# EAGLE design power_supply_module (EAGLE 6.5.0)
AUTHOR: N. Jackson; REV: A; TITLE: Power Supply Module

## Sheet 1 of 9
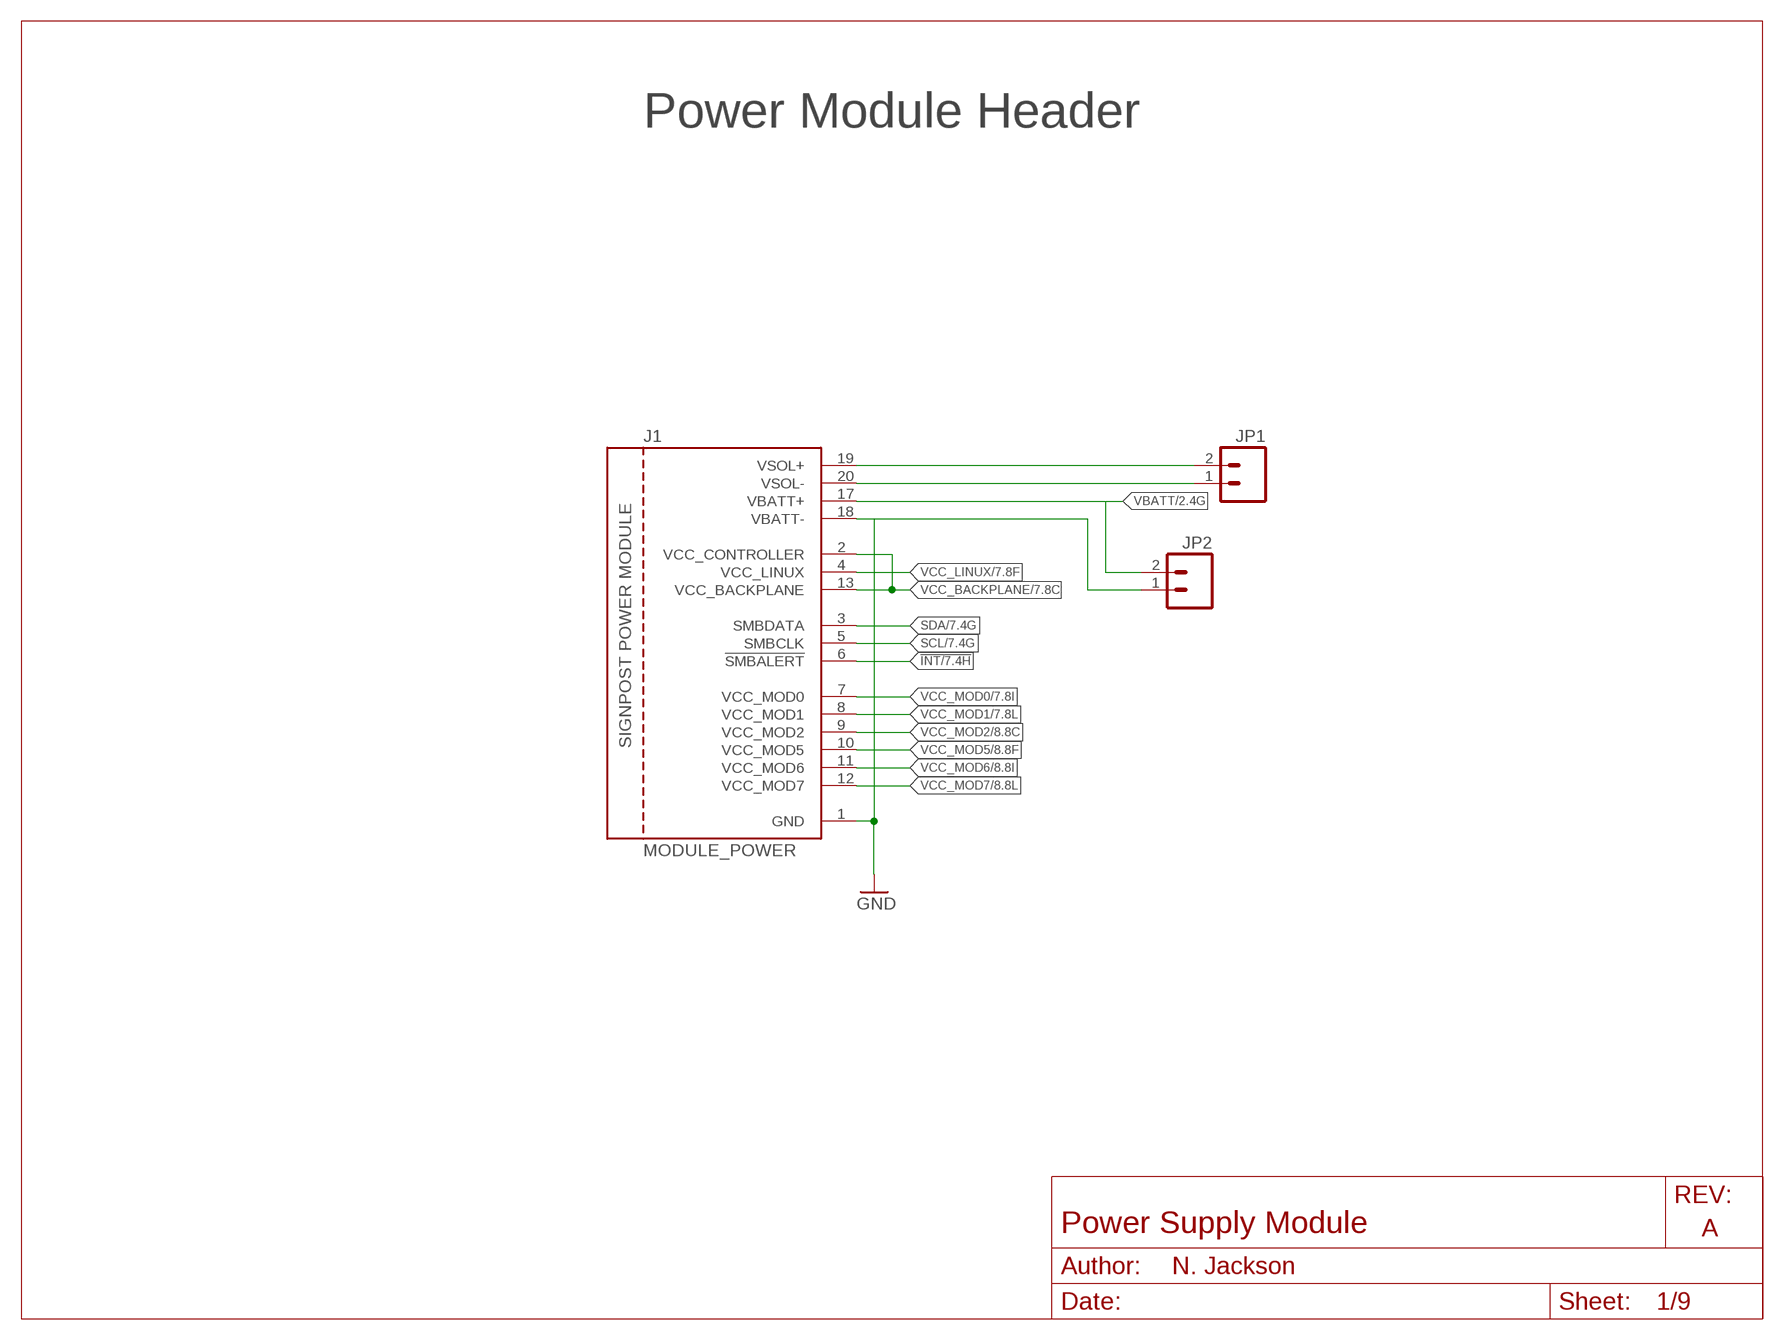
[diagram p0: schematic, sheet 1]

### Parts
J1  MODULE_POWER  [MODULE_POWER]
JP1  M02PTH  [1X02]
JP2  M02PTH  [1X02]

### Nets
!INT: J1.6(!SMBALERT) ; also sheet 7,8,9
GND: J1.1(GND) J1.18(VBATT-) JP2.1 ; also sheet 2,3,4,5,6,7,8,9
SCL: J1.5(SMBCLK) ; also sheet 7,8,9
SDA: J1.3(SMBDATA) ; also sheet 7,8,9
VBATT: J1.17(VBATT+) JP2.2 ; also sheet 2,3,4,5,6,9
VCC_BACKPLANE: J1.2(VCC_CONTROLLER) J1.13(VCC_BACKPLANE) ; also sheet 7,8,9
VCC_LINUX: J1.4(VCC_LINUX) ; also sheet 7,9
VCC_MOD0: J1.7(VCC_MOD0) ; also sheet 7,9
VCC_MOD1: J1.8(VCC_MOD1) ; also sheet 7,9
VCC_MOD2: J1.9(VCC_MOD2) ; also sheet 8,9
VCC_MOD5: J1.10(VCC_MOD5) ; also sheet 8,9
VCC_MOD6: J1.11(VCC_MOD6) ; also sheet 8,9
VCC_MOD7: J1.12(VCC_MOD7) ; also sheet 8,9
VSOL+: J1.19(VSOL+) JP1.2 ; also sheet 9
VSOL-: J1.20(VSOL-) JP1.1 ; also sheet 9

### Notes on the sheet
- Power Module Header

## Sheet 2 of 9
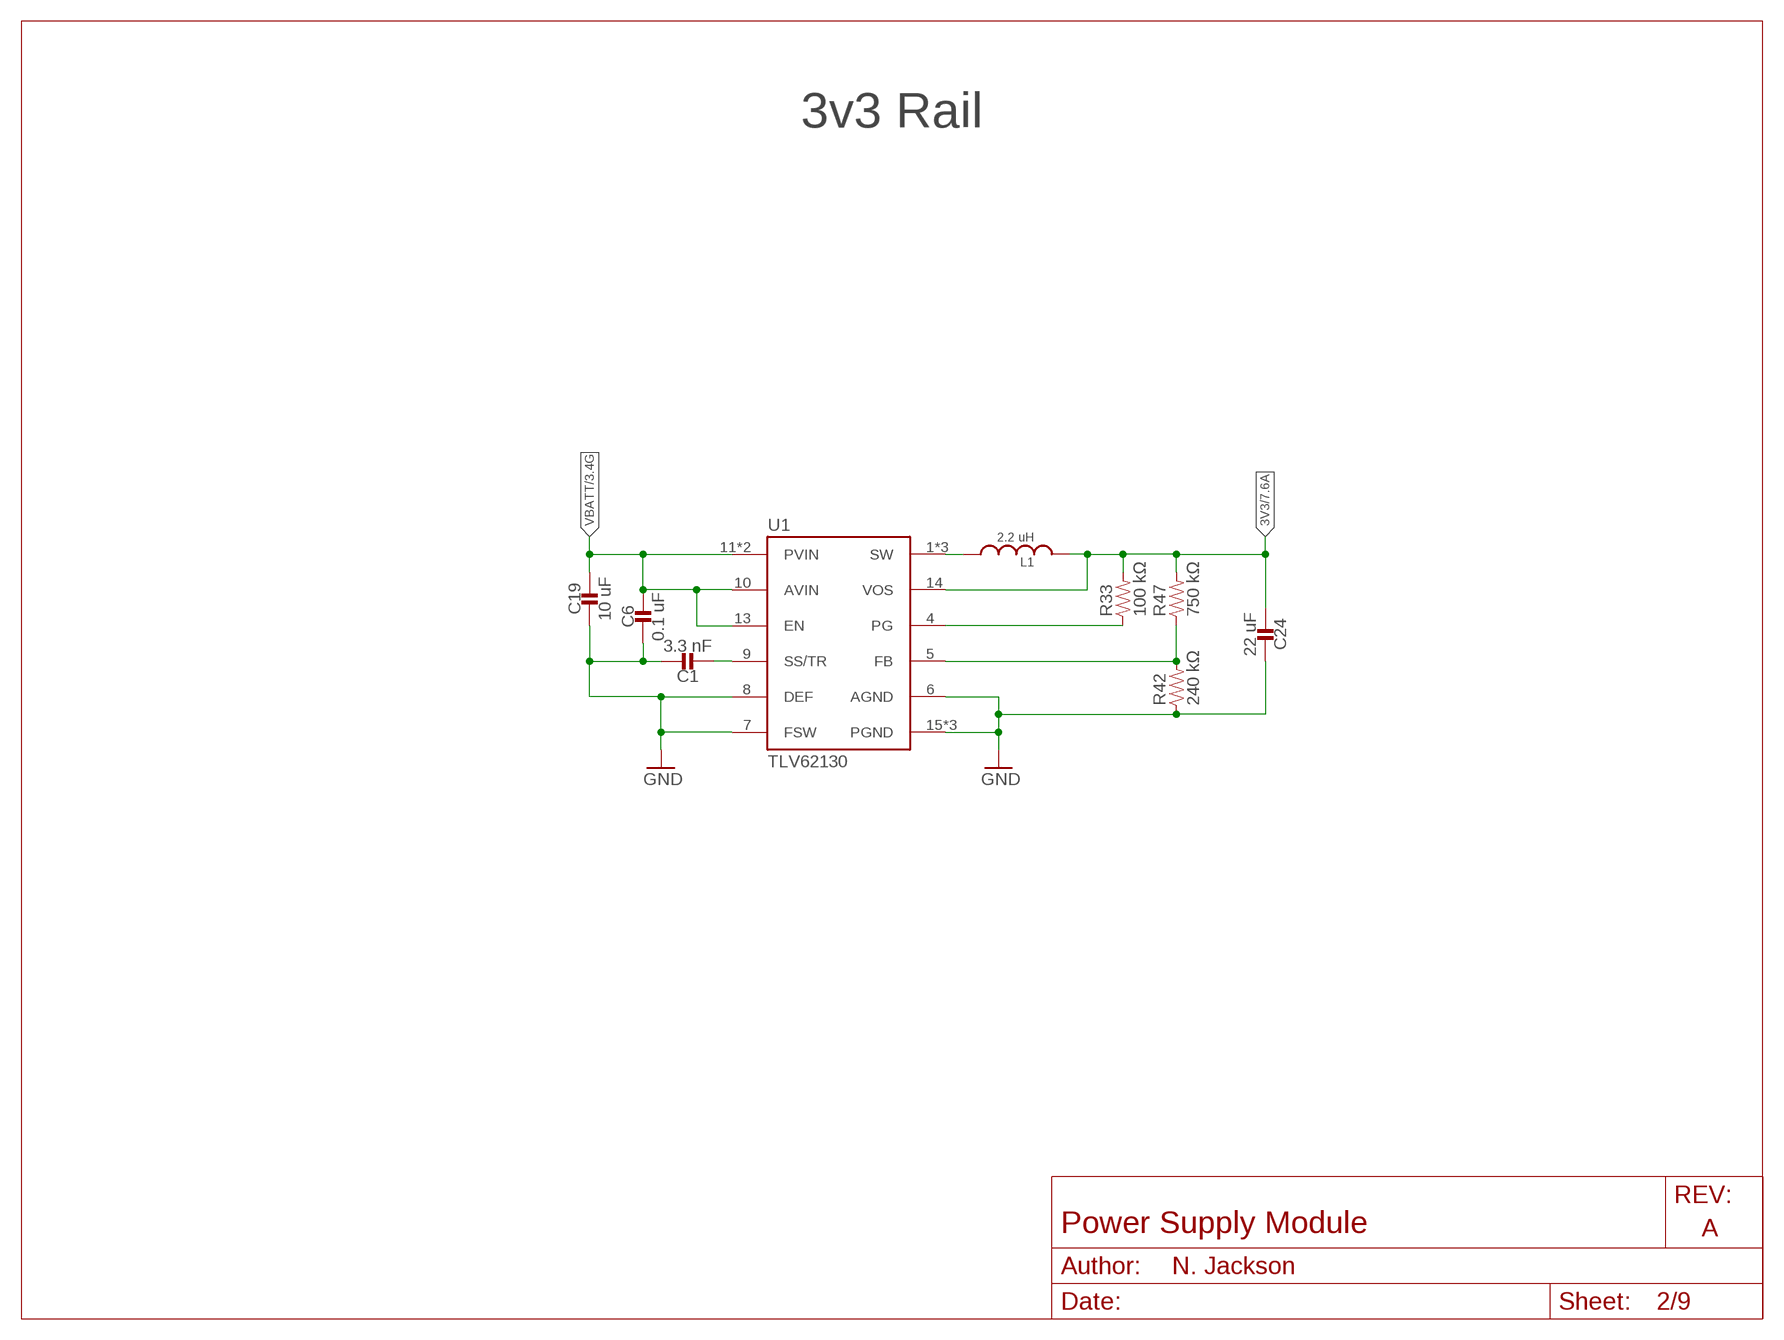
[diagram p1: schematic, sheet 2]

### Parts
C1  3.3 nF  CAPACITOR0402_CAP  [0402_CAP]
C6  0.1 uF  CAPACITOR0402_CAP  [0402_CAP]
C19  10 uF  CAPACITOR0805_CAP  [0805_CAP]
C24  22 uF  CAPACITOR0603_CAP  [0603_CAP]
L1  2.2 uH  INDUCTORIHL  [IHL-1212BZ-11]
R33  100 kΩ  RESISTOR0402_RES  [0402_RES]
R42  240 kΩ  RESISTOR0402_RES  [0402_RES]
R47  750 kΩ  RESISTOR0402_RES  [0402_RES]
U1  TLV62130  [TQFN-16/3MM]

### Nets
3V3: C24.2 L1.P$2 R33.2 R47.2 U1.14(VOS) ; also sheet 7,9
GND: C1.1 C6.2 C19.P$2 C24.1 R42.1 U1.6(AGND) U1.7(FSW) U1.8(DEF) U1.15(PGND) U1.16(PGND) U1.GND ; also sheet 1,3,4,5,6,7,8,9
N$61: C1.2 U1.9(SS/TR)
N$62: L1.P$1 U1.1(SW) U1.2(SW) U1.3(SW)
N$63: R33.1 U1.4(PG)
N$64: R42.2 R47.1 U1.5(FB)
VBATT: C6.1 C19.P$1 U1.10(AVIN) U1.11(PVIN) U1.12(PVIN) U1.13(EN) ; also sheet 1,3,4,5,6,9

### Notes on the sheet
- 3v3 Rail

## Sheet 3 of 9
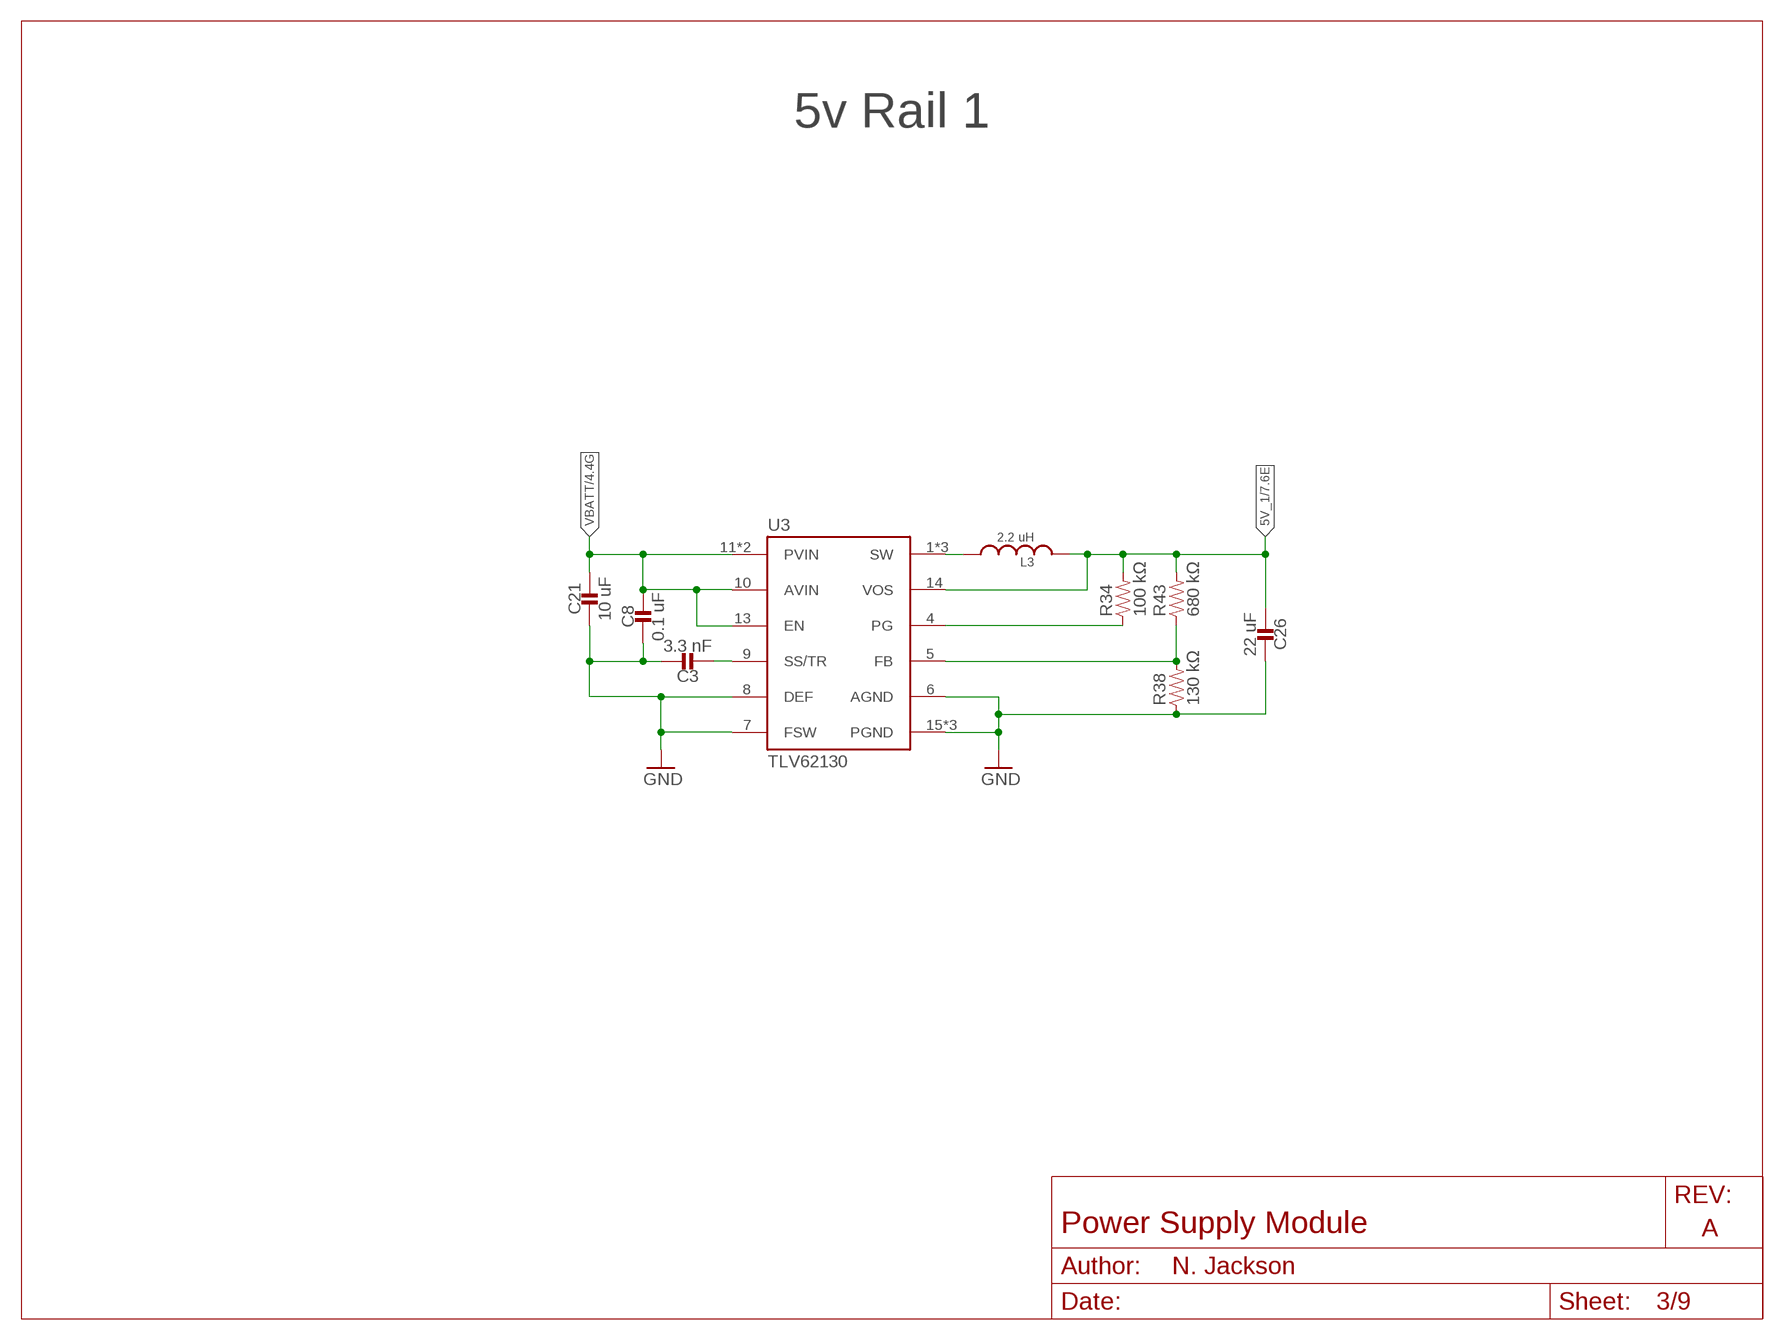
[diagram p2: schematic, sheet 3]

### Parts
C3  3.3 nF  CAPACITOR0402_CAP  [0402_CAP]
C8  0.1 uF  CAPACITOR0402_CAP  [0402_CAP]
C21  10 uF  CAPACITOR0805_CAP  [0805_CAP]
C26  22 uF  CAPACITOR0603_CAP  [0603_CAP]
L3  2.2 uH  INDUCTORIHL  [IHL-1212BZ-11]
R34  100 kΩ  RESISTOR0402_RES  [0402_RES]
R38  130 kΩ  RESISTOR0402_RES  [0402_RES]
R43  680 kΩ  RESISTOR0402_RES  [0402_RES]
U3  TLV62130  [TQFN-16/3MM]

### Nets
5V_1: C26.2 L3.P$2 R34.2 R43.2 U3.14(VOS) ; also sheet 7,9
GND: C3.1 C8.2 C21.P$2 C26.1 R38.1 U3.6(AGND) U3.7(FSW) U3.8(DEF) U3.15(PGND) U3.16(PGND) U3.GND ; also sheet 1,2,4,5,6,7,8,9
N$5: C3.2 U3.9(SS/TR)
N$6: L3.P$1 U3.1(SW) U3.2(SW) U3.3(SW)
N$7: R34.1 U3.4(PG)
N$9: R38.2 R43.1 U3.5(FB)
VBATT: C8.1 C21.P$1 U3.10(AVIN) U3.11(PVIN) U3.12(PVIN) U3.13(EN) ; also sheet 1,2,4,5,6,9

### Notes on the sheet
- 5v Rail 1

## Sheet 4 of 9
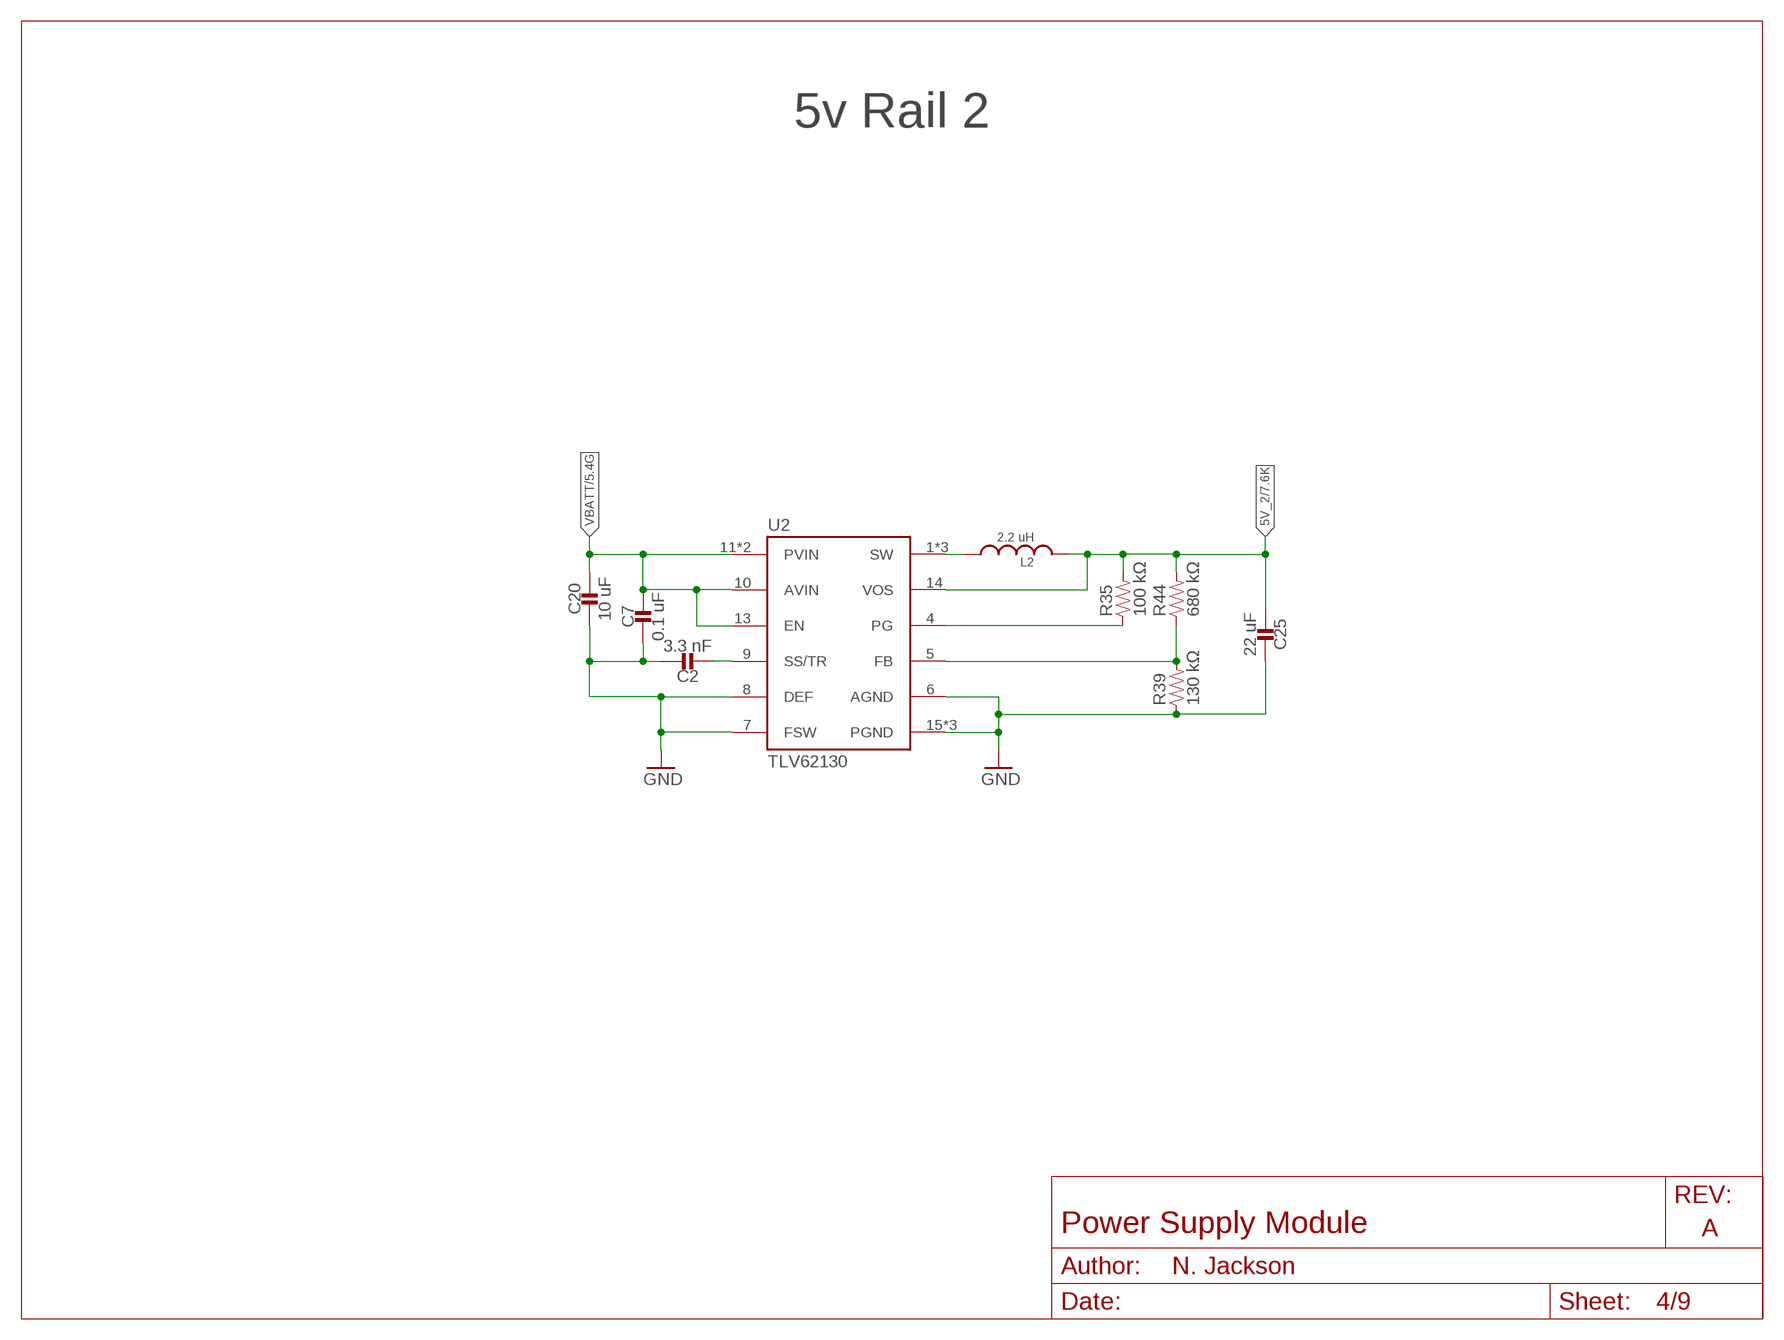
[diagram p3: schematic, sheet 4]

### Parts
C2  3.3 nF  CAPACITOR0402_CAP  [0402_CAP]
C7  0.1 uF  CAPACITOR0402_CAP  [0402_CAP]
C20  10 uF  CAPACITOR0805_CAP  [0805_CAP]
C25  22 uF  CAPACITOR0603_CAP  [0603_CAP]
L2  2.2 uH  INDUCTORIHL  [IHL-1212BZ-11]
R35  100 kΩ  RESISTOR0402_RES  [0402_RES]
R39  130 kΩ  RESISTOR0402_RES  [0402_RES]
R44  680 kΩ  RESISTOR0402_RES  [0402_RES]
U2  TLV62130  [TQFN-16/3MM]

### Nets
5V_2: C25.2 L2.P$2 R35.2 R44.2 U2.14(VOS) ; also sheet 7,9
GND: C2.1 C7.2 C20.P$2 C25.1 R39.1 U2.6(AGND) U2.7(FSW) U2.8(DEF) U2.15(PGND) U2.16(PGND) U2.GND ; also sheet 1,2,3,5,6,7,8,9
N$1: C2.2 U2.9(SS/TR)
N$2: L2.P$1 U2.1(SW) U2.2(SW) U2.3(SW)
N$3: R35.1 U2.4(PG)
N$4: R39.2 R44.1 U2.5(FB)
VBATT: C7.1 C20.P$1 U2.10(AVIN) U2.11(PVIN) U2.12(PVIN) U2.13(EN) ; also sheet 1,2,3,5,6,9

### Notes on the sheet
- 5v Rail 2

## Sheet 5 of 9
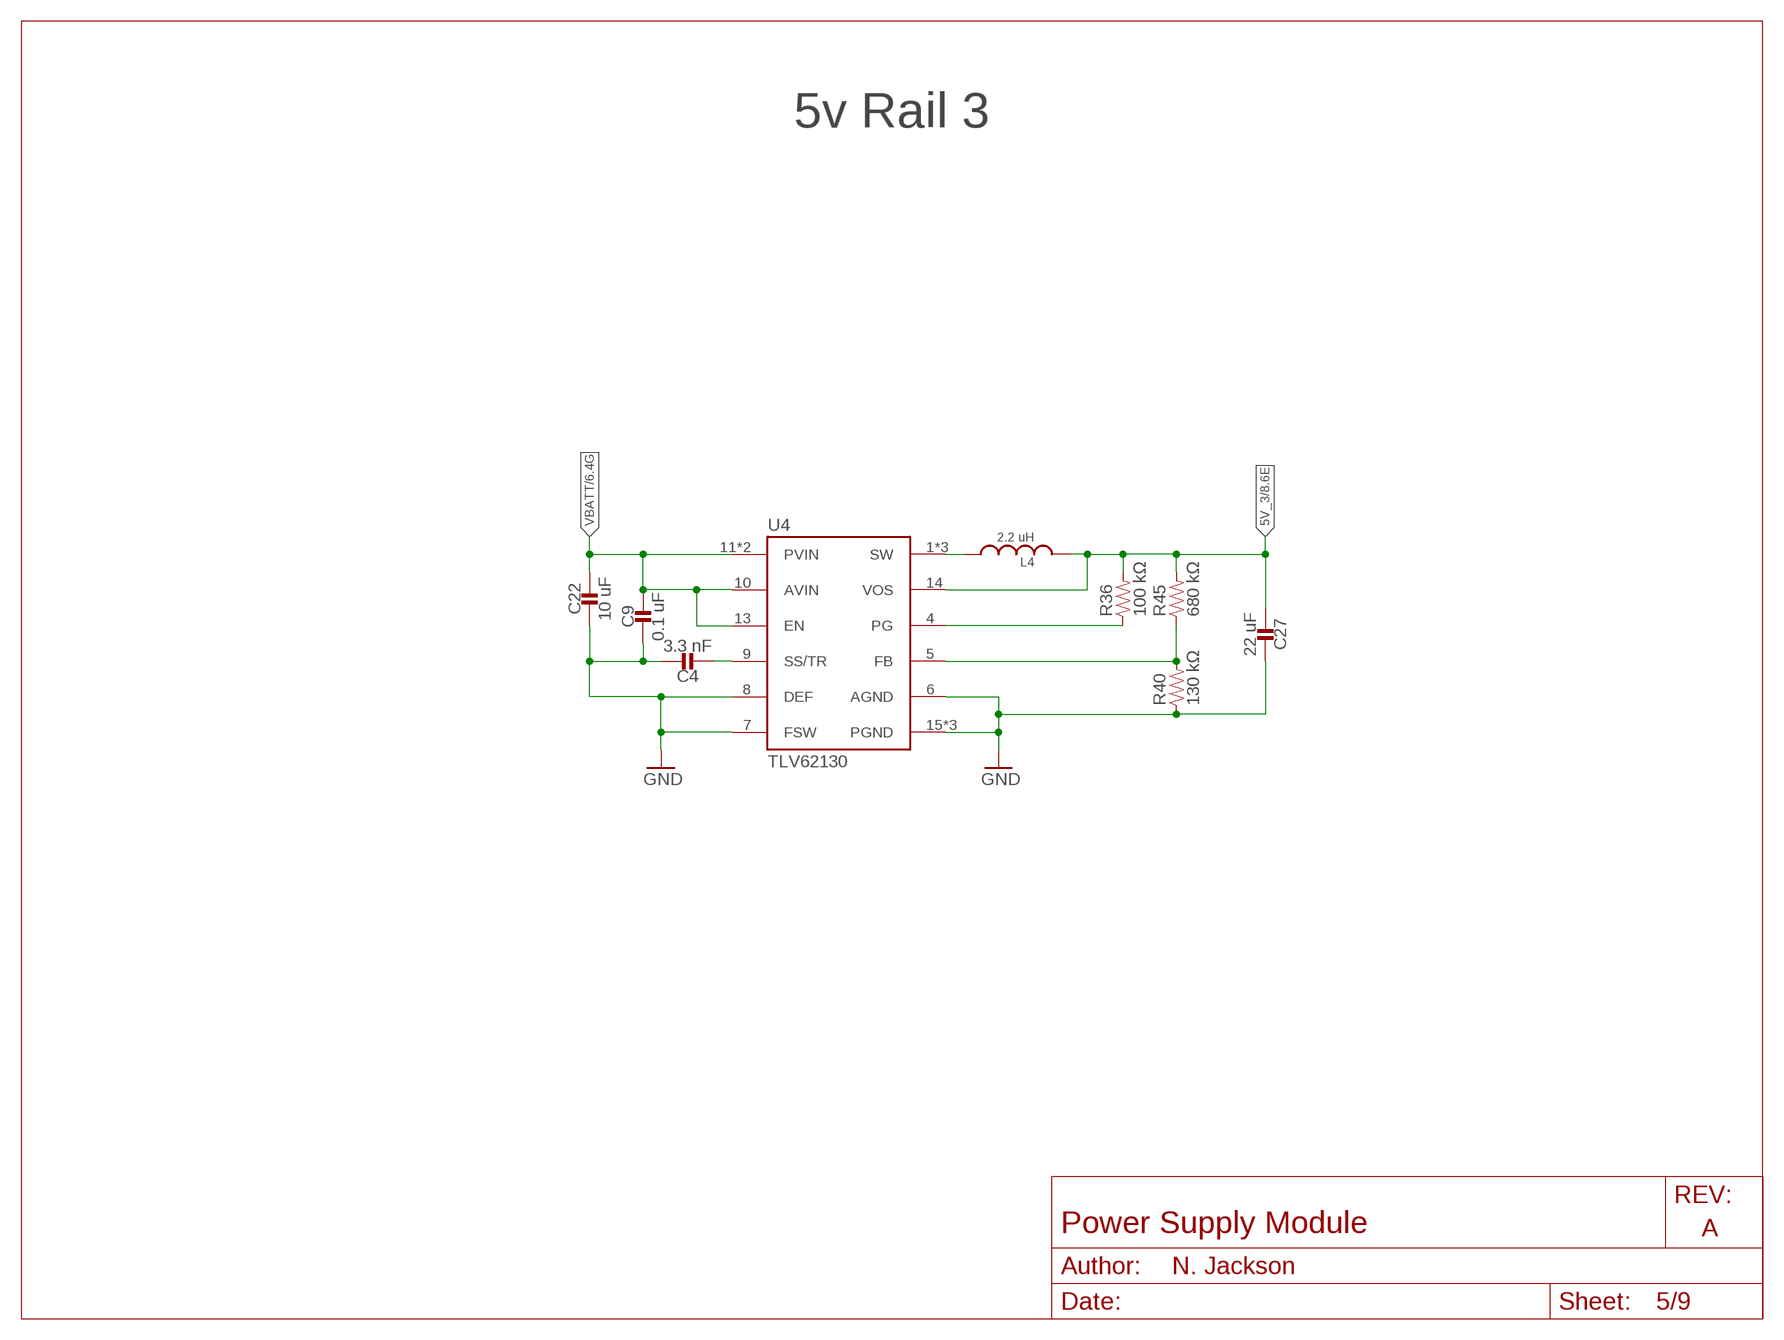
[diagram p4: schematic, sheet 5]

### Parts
C4  3.3 nF  CAPACITOR0402_CAP  [0402_CAP]
C9  0.1 uF  CAPACITOR0402_CAP  [0402_CAP]
C22  10 uF  CAPACITOR0805_CAP  [0805_CAP]
C27  22 uF  CAPACITOR0603_CAP  [0603_CAP]
L4  2.2 uH  INDUCTORIHL  [IHL-1212BZ-11]
R36  100 kΩ  RESISTOR0402_RES  [0402_RES]
R40  130 kΩ  RESISTOR0402_RES  [0402_RES]
R45  680 kΩ  RESISTOR0402_RES  [0402_RES]
U4  TLV62130  [TQFN-16/3MM]

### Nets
5V_3: C27.2 L4.P$2 R36.2 R45.2 U4.14(VOS) ; also sheet 8,9
GND: C4.1 C9.2 C22.P$2 C27.1 R40.1 U4.6(AGND) U4.7(FSW) U4.8(DEF) U4.15(PGND) U4.16(PGND) U4.GND ; also sheet 1,2,3,4,6,7,8,9
N$8: C4.2 U4.9(SS/TR)
N$10: L4.P$1 U4.1(SW) U4.2(SW) U4.3(SW)
N$11: R36.1 U4.4(PG)
N$12: R40.2 R45.1 U4.5(FB)
VBATT: C9.1 C22.P$1 U4.10(AVIN) U4.11(PVIN) U4.12(PVIN) U4.13(EN) ; also sheet 1,2,3,4,6,9

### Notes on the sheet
- 5v Rail 3

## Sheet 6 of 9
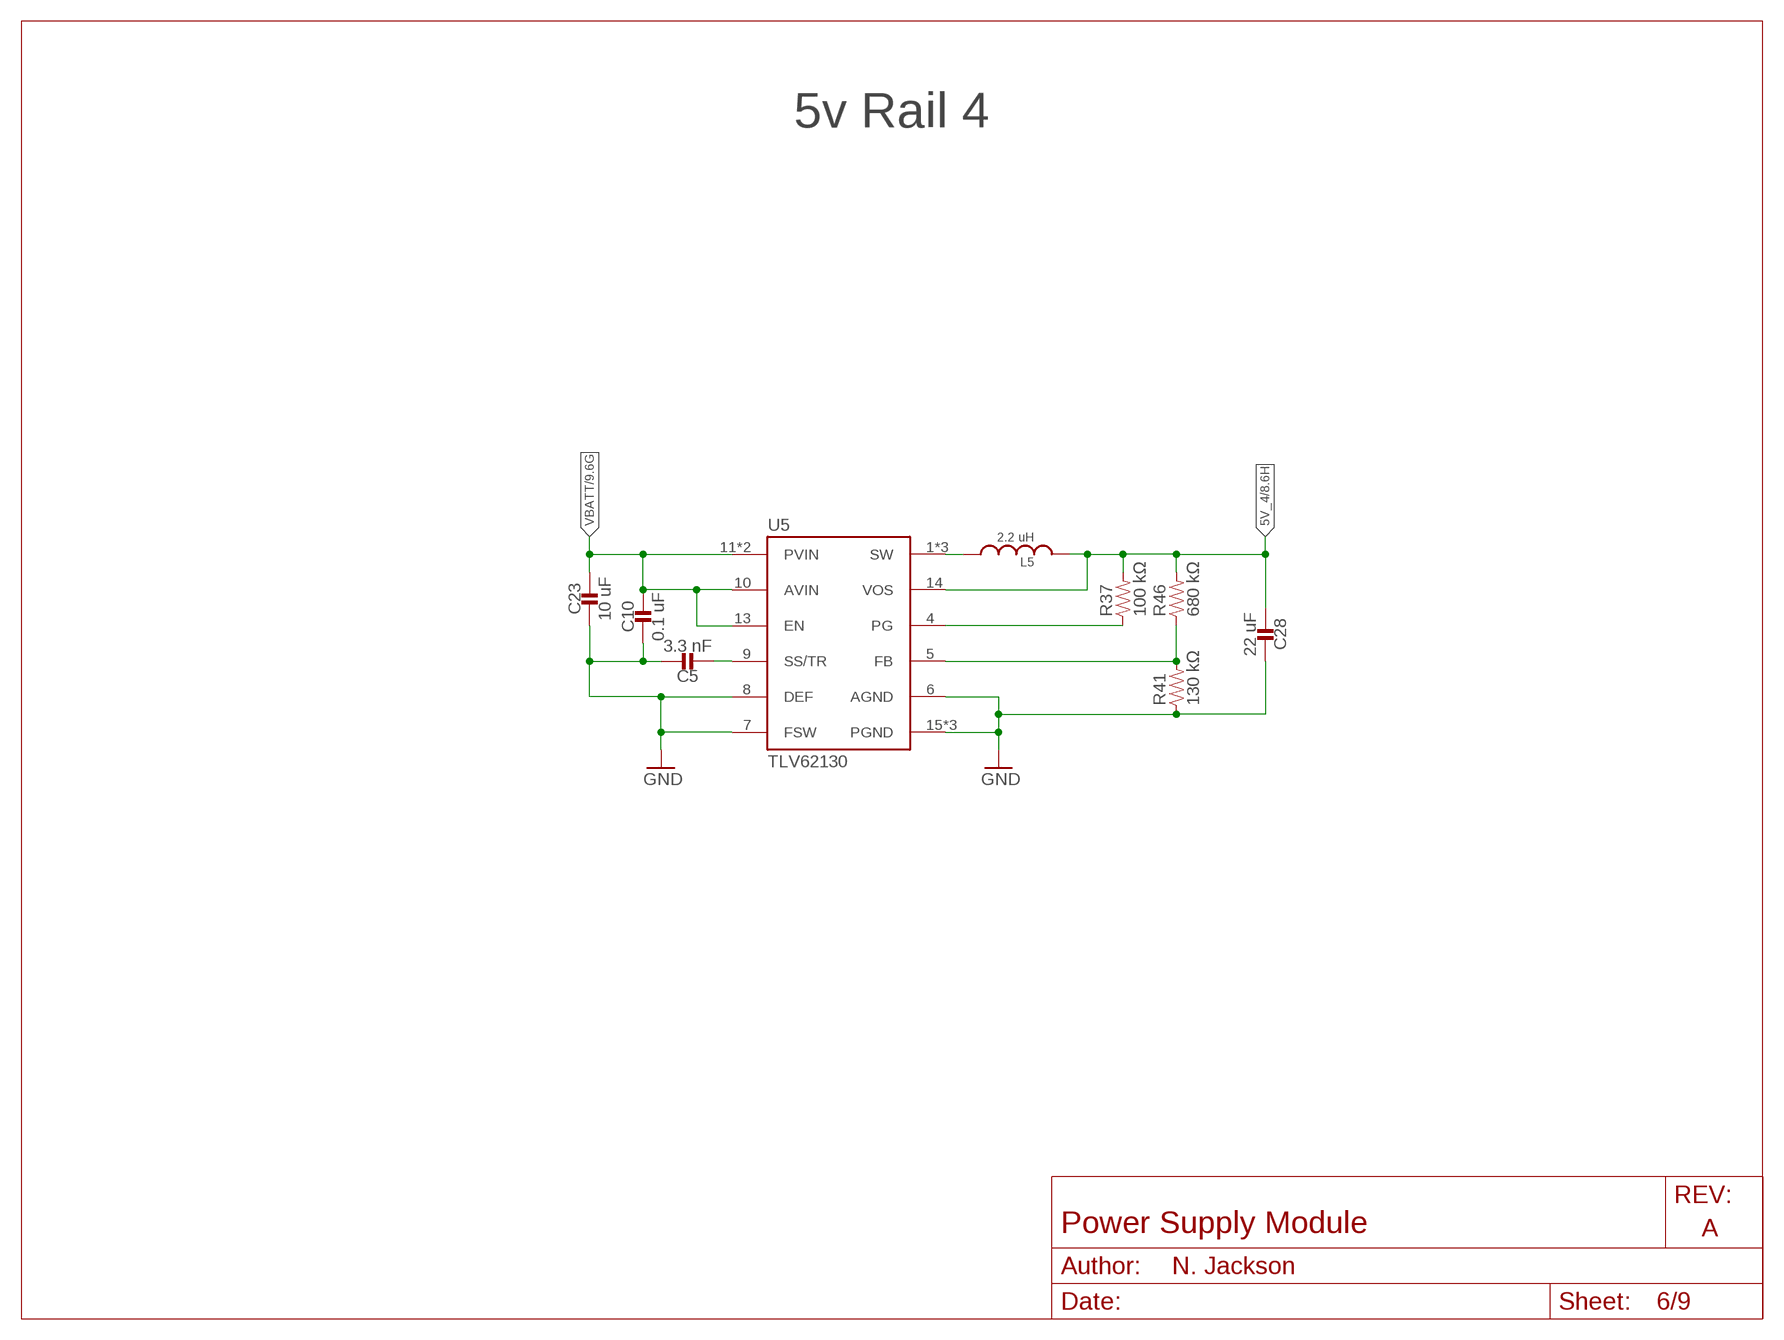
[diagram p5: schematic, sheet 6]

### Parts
C5  3.3 nF  CAPACITOR0402_CAP  [0402_CAP]
C10  0.1 uF  CAPACITOR0402_CAP  [0402_CAP]
C23  10 uF  CAPACITOR0805_CAP  [0805_CAP]
C28  22 uF  CAPACITOR0603_CAP  [0603_CAP]
L5  2.2 uH  INDUCTORIHL  [IHL-1212BZ-11]
R37  100 kΩ  RESISTOR0402_RES  [0402_RES]
R41  130 kΩ  RESISTOR0402_RES  [0402_RES]
R46  680 kΩ  RESISTOR0402_RES  [0402_RES]
U5  TLV62130  [TQFN-16/3MM]

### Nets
5V_4: C28.2 L5.P$2 R37.2 R46.2 U5.14(VOS) ; also sheet 8,9
GND: C5.1 C10.2 C23.P$2 C28.1 R41.1 U5.6(AGND) U5.7(FSW) U5.8(DEF) U5.15(PGND) U5.16(PGND) U5.GND ; also sheet 1,2,3,4,5,7,8,9
N$13: C5.2 U5.9(SS/TR)
N$14: L5.P$1 U5.1(SW) U5.2(SW) U5.3(SW)
N$15: R37.1 U5.4(PG)
N$16: R41.2 R46.1 U5.5(FB)
VBATT: C10.1 C23.P$1 U5.10(AVIN) U5.11(PVIN) U5.12(PVIN) U5.13(EN) ; also sheet 1,2,3,4,5,9

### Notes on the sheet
- 5v Rail 4

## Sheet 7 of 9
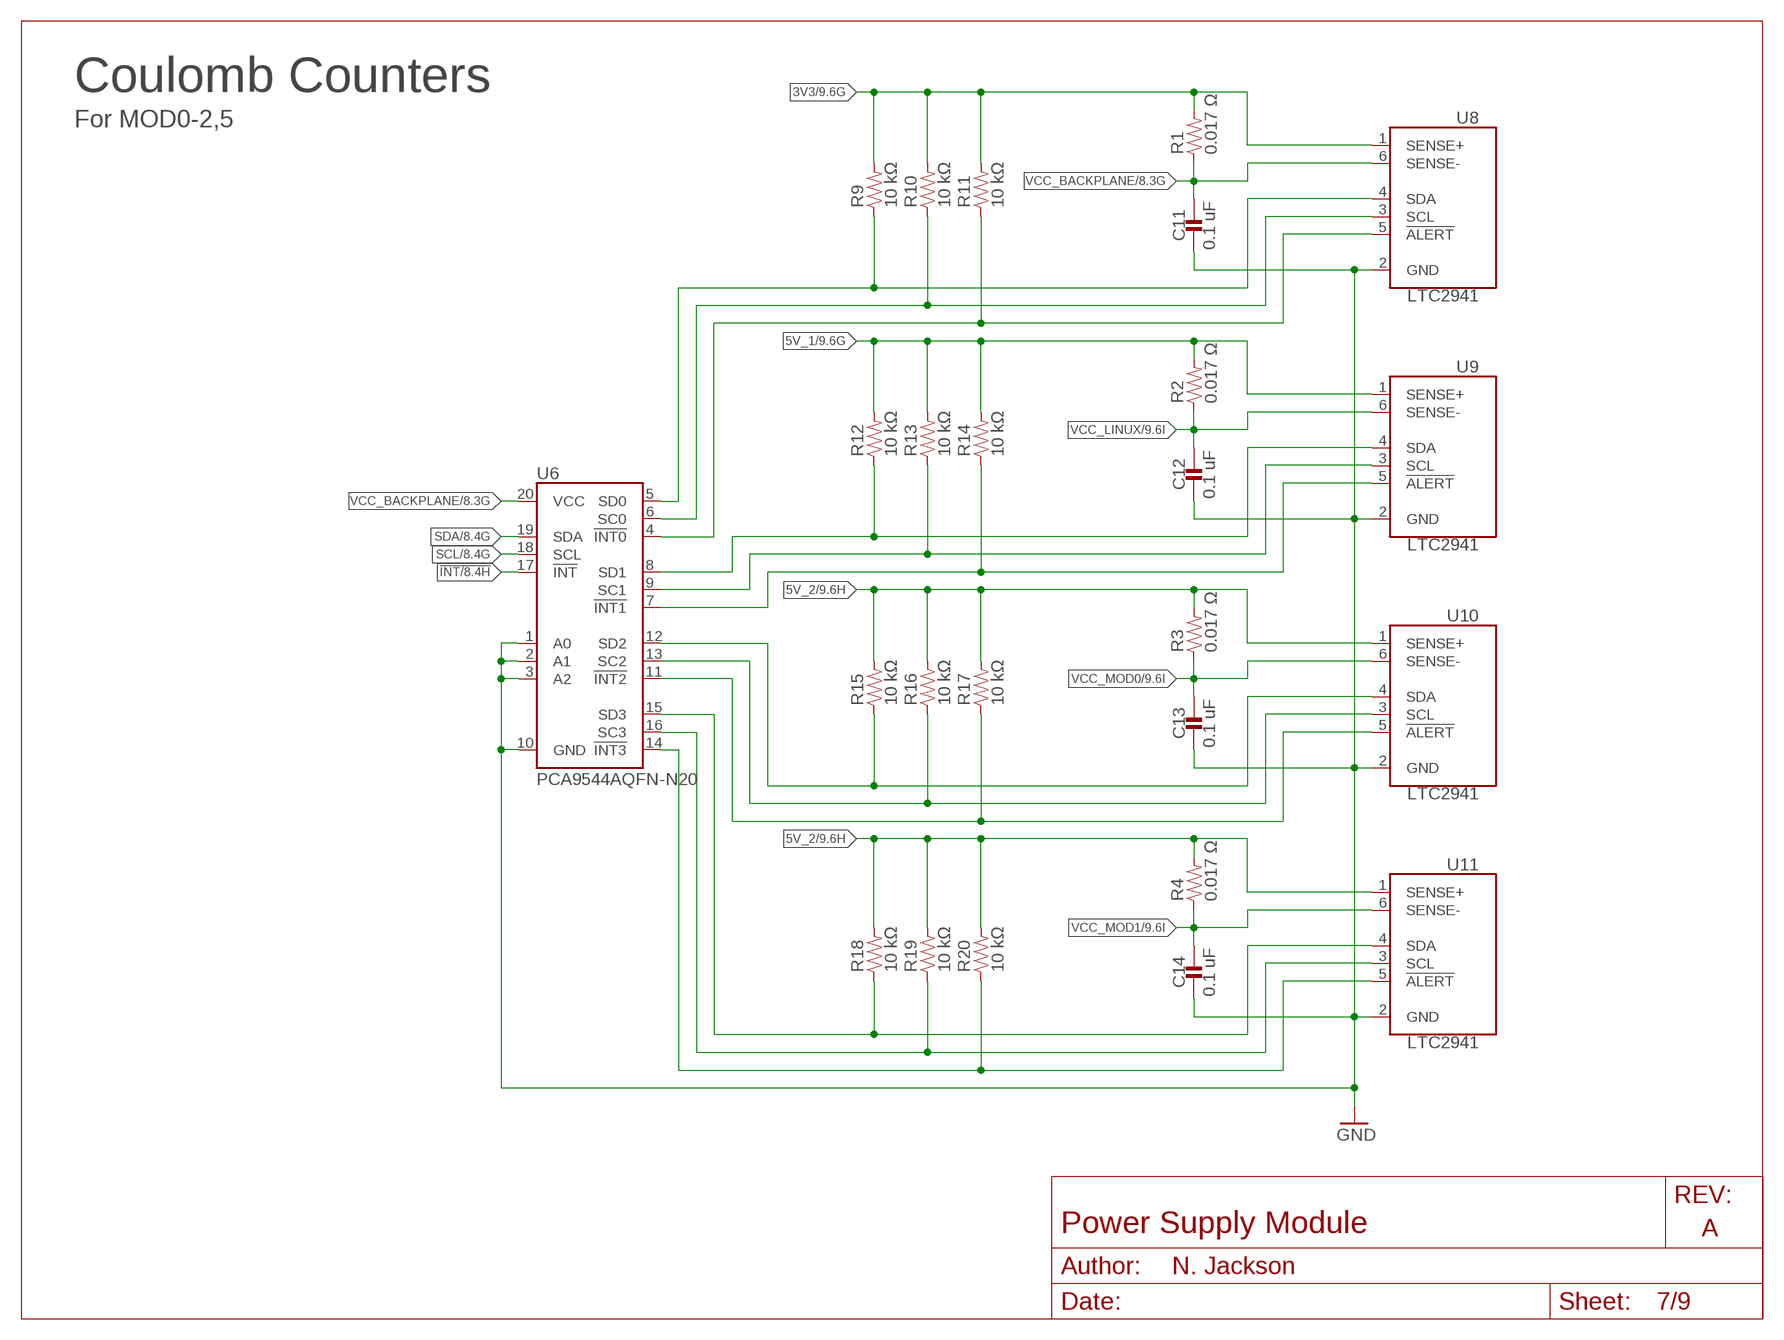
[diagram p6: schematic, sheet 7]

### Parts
C11  0.1 uF  CAPACITOR0402_CAP  [0402_CAP]
C12  0.1 uF  CAPACITOR0402_CAP  [0402_CAP]
C13  0.1 uF  CAPACITOR0402_CAP  [0402_CAP]
C14  0.1 uF  CAPACITOR0402_CAP  [0402_CAP]
R1  0.017 Ω  RESISTOR0805_RES  [0805_RES]
R2  0.017 Ω  RESISTOR0805_RES  [0805_RES]
R3  0.017 Ω  RESISTOR0805_RES  [0805_RES]
R4  0.017 Ω  RESISTOR0805_RES  [0805_RES]
R9  10 kΩ  RESISTOR0402_RES  [0402_RES]
R10  10 kΩ  RESISTOR0402_RES  [0402_RES]
R11  10 kΩ  RESISTOR0402_RES  [0402_RES]
R12  10 kΩ  RESISTOR0402_RES  [0402_RES]
R13  10 kΩ  RESISTOR0402_RES  [0402_RES]
R14  10 kΩ  RESISTOR0402_RES  [0402_RES]
R15  10 kΩ  RESISTOR0402_RES  [0402_RES]
R16  10 kΩ  RESISTOR0402_RES  [0402_RES]
R17  10 kΩ  RESISTOR0402_RES  [0402_RES]
R18  10 kΩ  RESISTOR0402_RES  [0402_RES]
R19  10 kΩ  RESISTOR0402_RES  [0402_RES]
R20  10 kΩ  RESISTOR0402_RES  [0402_RES]
U6  PCA9544AQFN-N20  [QFN-N20]
U8  LTC2941  [DFN-6-2MMX3MM]
U9  LTC2941  [DFN-6-2MMX3MM]
U10  LTC2941  [DFN-6-2MMX3MM]
U11  LTC2941  [DFN-6-2MMX3MM]

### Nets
3V3: R1.2 R9.2 R10.2 R11.2 U8.1(SENSE+) ; also sheet 2,9
5V_1: R2.2 R12.2 R13.2 R14.2 U9.1(SENSE+) ; also sheet 3,9
5V_2: R3.2 R4.2 R15.2 R16.2 R17.2 R18.2 R19.2 R20.2 U10.1(SENSE+) U11.1(SENSE+) ; also sheet 4,9
!INT: U6.17(!INT) ; also sheet 1,8,9
GND: C11.2 C12.2 C13.2 C14.2 U6.1(A0) U6.2(A1) U6.3(A2) U6.10(GND) U8.2(GND) U9.2(GND) U10.2(GND) U11.2(GND) ; also sheet 1,2,3,4,5,6,8,9
N$43: R9.1 U6.5(SD0) U8.4(SDA)
N$47: R10.1 U6.6(SC0) U8.3(SCL)
N$52: R15.1 U6.12(SD2) U10.4(SDA)
N$53: R16.1 U6.13(SC2) U10.3(SCL)
N$54: R17.1 U6.11(!INT2) U10.5(!ALERT)
N$55: R18.1 U6.15(SD3) U11.4(SDA)
N$56: R19.1 U6.16(SC3) U11.3(SCL)
N$57: R20.1 U6.14(!INT3) U11.5(!ALERT)
N$67: R11.1 U6.4(!INT0) U8.5(!ALERT)
N$68: R12.1 U6.8(SD1) U9.4(SDA)
N$70: R13.1 U6.9(SC1) U9.3(SCL)
N$71: R14.1 U6.7(!INT1) U9.5(!ALERT)
SCL: U6.18(SCL) ; also sheet 1,8,9
SDA: U6.19(SDA) ; also sheet 1,8,9
VCC_BACKPLANE: C11.1 R1.1 U6.20(VCC) U8.6(SENSE-) ; also sheet 1,8,9
VCC_LINUX: C12.1 R2.1 U9.6(SENSE-) ; also sheet 1,9
VCC_MOD0: C13.1 R3.1 U10.6(SENSE-) ; also sheet 1,9
VCC_MOD1: C14.1 R4.1 U11.6(SENSE-) ; also sheet 1,9

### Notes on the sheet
- Coulomb Counters
- For MOD0-2,5

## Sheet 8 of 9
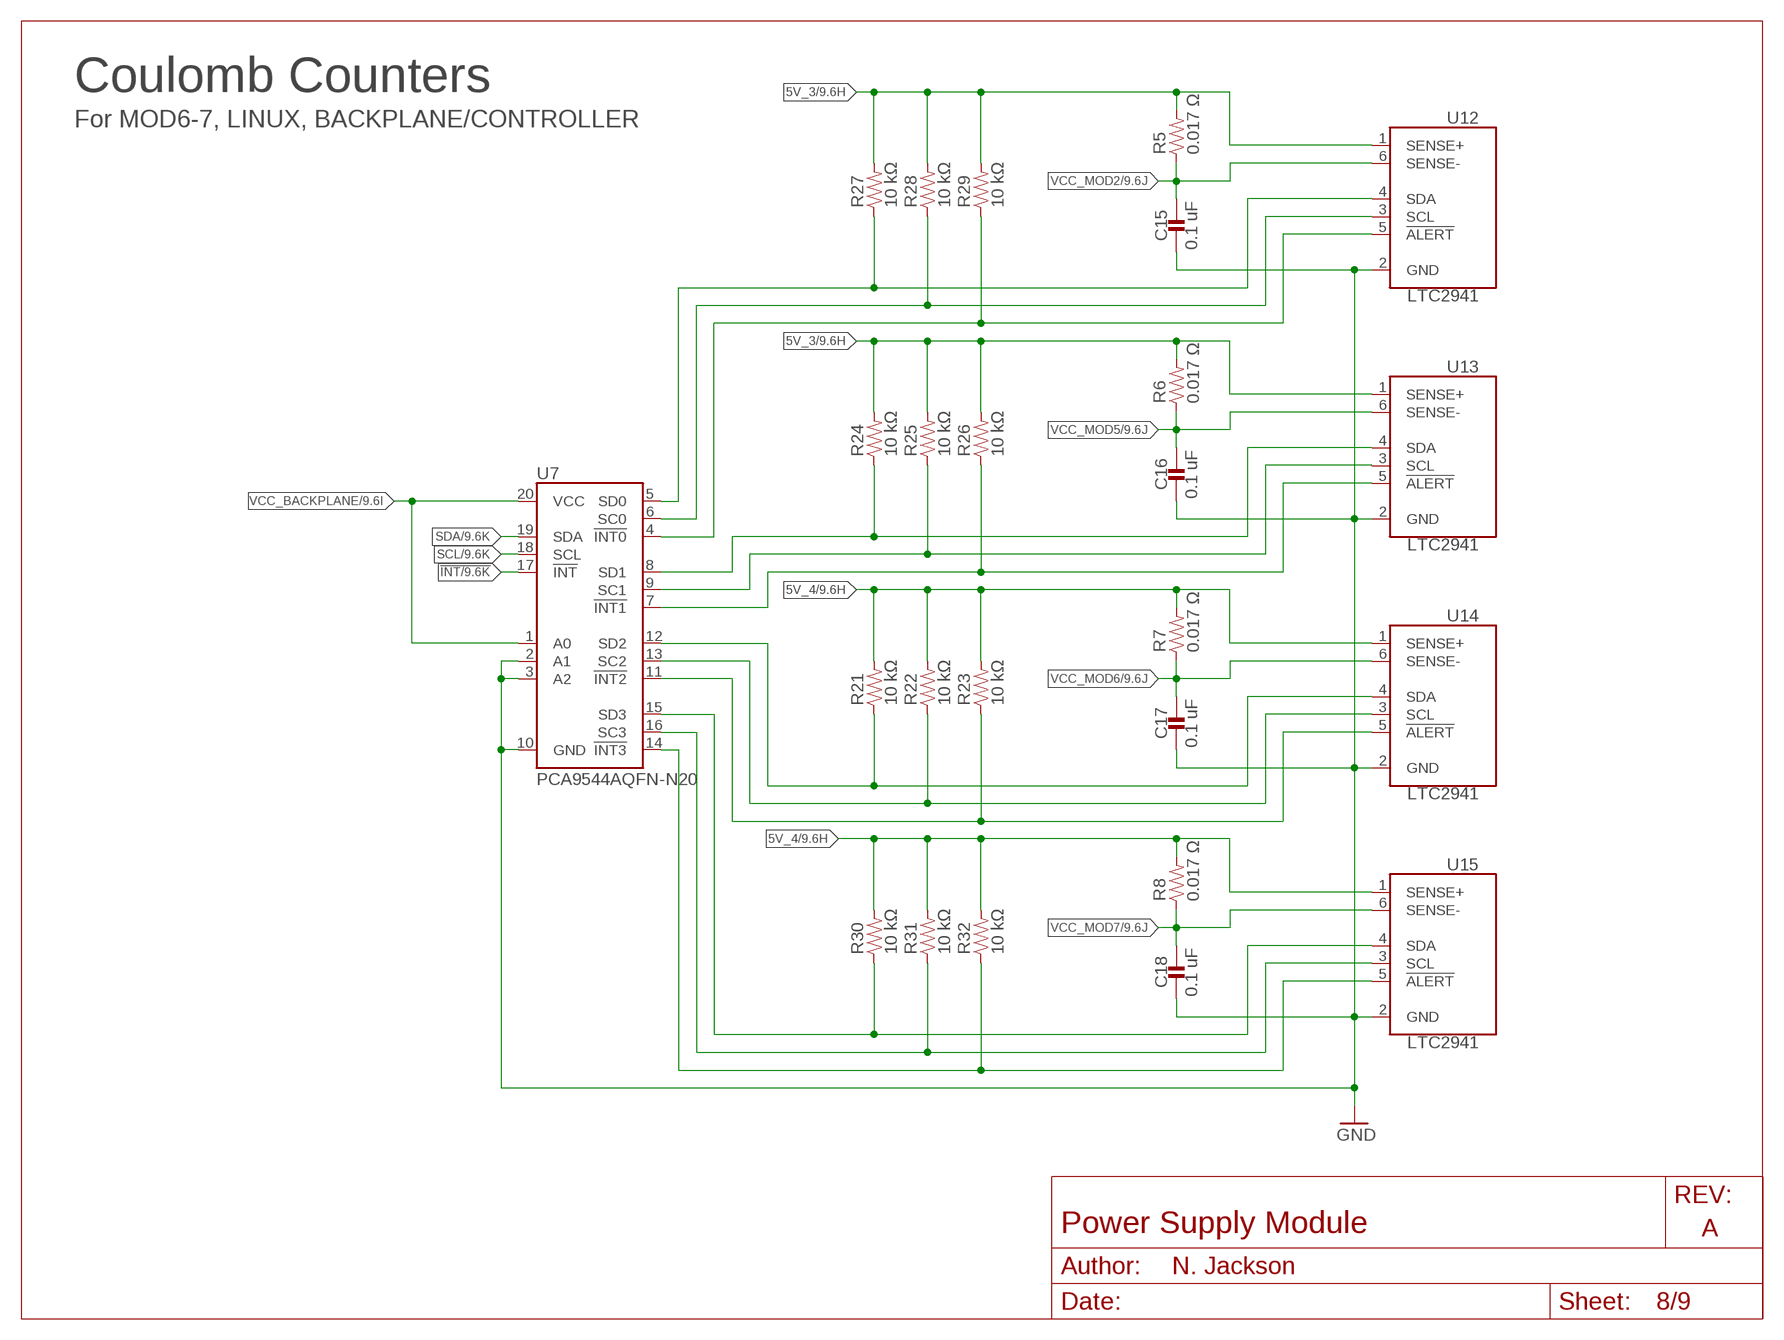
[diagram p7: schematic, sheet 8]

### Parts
C15  0.1 uF  CAPACITOR0402_CAP  [0402_CAP]
C16  0.1 uF  CAPACITOR0402_CAP  [0402_CAP]
C17  0.1 uF  CAPACITOR0402_CAP  [0402_CAP]
C18  0.1 uF  CAPACITOR0402_CAP  [0402_CAP]
R5  0.017 Ω  RESISTOR0805_RES  [0805_RES]
R6  0.017 Ω  RESISTOR0805_RES  [0805_RES]
R7  0.017 Ω  RESISTOR0805_RES  [0805_RES]
R8  0.017 Ω  RESISTOR0805_RES  [0805_RES]
R21  10 kΩ  RESISTOR0402_RES  [0402_RES]
R22  10 kΩ  RESISTOR0402_RES  [0402_RES]
R23  10 kΩ  RESISTOR0402_RES  [0402_RES]
R24  10 kΩ  RESISTOR0402_RES  [0402_RES]
R25  10 kΩ  RESISTOR0402_RES  [0402_RES]
R26  10 kΩ  RESISTOR0402_RES  [0402_RES]
R27  10 kΩ  RESISTOR0402_RES  [0402_RES]
R28  10 kΩ  RESISTOR0402_RES  [0402_RES]
R29  10 kΩ  RESISTOR0402_RES  [0402_RES]
R30  10 kΩ  RESISTOR0402_RES  [0402_RES]
R31  10 kΩ  RESISTOR0402_RES  [0402_RES]
R32  10 kΩ  RESISTOR0402_RES  [0402_RES]
U7  PCA9544AQFN-N20  [QFN-N20]
U12  LTC2941  [DFN-6-2MMX3MM]
U13  LTC2941  [DFN-6-2MMX3MM]
U14  LTC2941  [DFN-6-2MMX3MM]
U15  LTC2941  [DFN-6-2MMX3MM]

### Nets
5V_3: R5.2 R6.2 R24.2 R25.2 R26.2 R27.2 R28.2 R29.2 U12.1(SENSE+) U13.1(SENSE+) ; also sheet 5,9
5V_4: R7.2 R8.2 R21.2 R22.2 R23.2 R30.2 R31.2 R32.2 U14.1(SENSE+) U15.1(SENSE+) ; also sheet 6,9
!INT: U7.17(!INT) ; also sheet 1,7,9
GND: C15.2 C16.2 C17.2 C18.2 U7.2(A1) U7.3(A2) U7.10(GND) U12.2(GND) U13.2(GND) U14.2(GND) U15.2(GND) ; also sheet 1,2,3,4,5,6,7,9
N$21: R27.1 U7.5(SD0) U12.4(SDA)
N$22: R28.1 U7.6(SC0) U12.3(SCL)
N$23: R21.1 U7.12(SD2) U14.4(SDA)
N$24: R22.1 U7.13(SC2) U14.3(SCL)
N$25: R23.1 U7.11(!INT2) U14.5(!ALERT)
N$26: R30.1 U7.15(SD3) U15.4(SDA)
N$27: R31.1 U7.16(SC3) U15.3(SCL)
N$46: R32.1 U7.14(!INT3) U15.5(!ALERT)
N$48: R29.1 U7.4(!INT0) U12.5(!ALERT)
N$49: R24.1 U7.8(SD1) U13.4(SDA)
N$50: R25.1 U7.9(SC1) U13.3(SCL)
N$51: R26.1 U7.7(!INT1) U13.5(!ALERT)
SCL: U7.18(SCL) ; also sheet 1,7,9
SDA: U7.19(SDA) ; also sheet 1,7,9
VCC_BACKPLANE: U7.1(A0) U7.20(VCC) ; also sheet 1,7,9
VCC_MOD2: C15.1 R5.1 U12.6(SENSE-) ; also sheet 1,9
VCC_MOD5: C16.1 R6.1 U13.6(SENSE-) ; also sheet 1,9
VCC_MOD6: C17.1 R7.1 U14.6(SENSE-) ; also sheet 1,9
VCC_MOD7: C18.1 R8.1 U15.6(SENSE-) ; also sheet 1,9

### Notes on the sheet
- Coulomb Counters
- For MOD6-7, LINUX, BACKPLANE/CONTROLLER

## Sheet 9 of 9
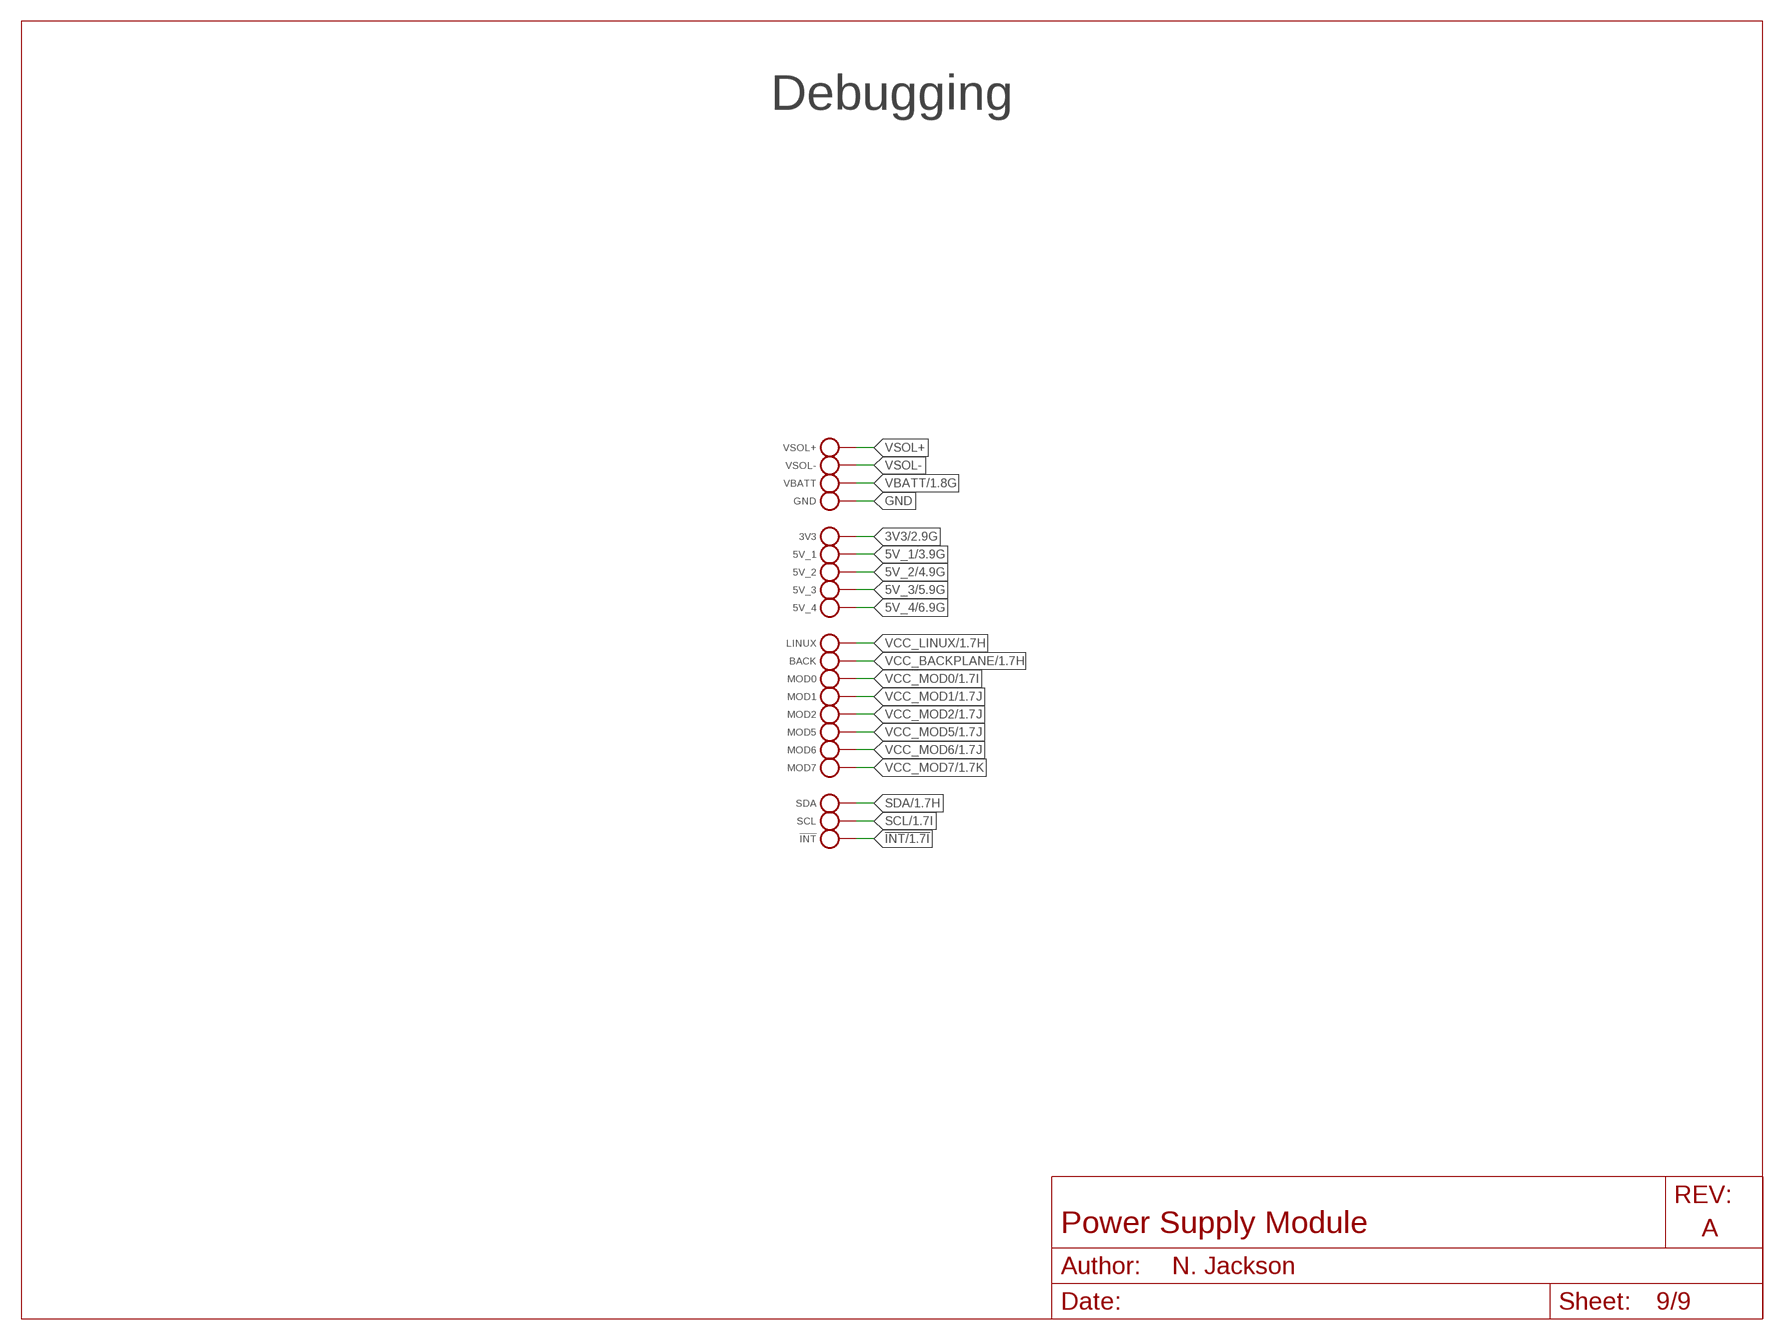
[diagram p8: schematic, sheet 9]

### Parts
3V3  TEST_POINT_0.040IN  [TESTPOINT_0.040IN]
5V_1  TEST_POINT_0.040IN  [TESTPOINT_0.040IN]
5V_2  TEST_POINT_0.040IN  [TESTPOINT_0.040IN]
5V_3  TEST_POINT_0.040IN  [TESTPOINT_0.040IN]
5V_4  TEST_POINT_0.040IN  [TESTPOINT_0.040IN]
!INT  TEST_POINT_0.040IN  [TESTPOINT_0.040IN]
BACK  TEST_POINT_0.040IN  [TESTPOINT_0.040IN]
GND  TEST_POINT_0.040IN  [TESTPOINT_0.040IN]
LINUX  TEST_POINT_0.040IN  [TESTPOINT_0.040IN]
MOD0  TEST_POINT_0.040IN  [TESTPOINT_0.040IN]
MOD1  TEST_POINT_0.040IN  [TESTPOINT_0.040IN]
MOD2  TEST_POINT_0.040IN  [TESTPOINT_0.040IN]
MOD5  TEST_POINT_0.040IN  [TESTPOINT_0.040IN]
MOD6  TEST_POINT_0.040IN  [TESTPOINT_0.040IN]
MOD7  TEST_POINT_0.040IN  [TESTPOINT_0.040IN]
SCL  TEST_POINT_0.040IN  [TESTPOINT_0.040IN]
SDA  TEST_POINT_0.040IN  [TESTPOINT_0.040IN]
VBATT  TEST_POINT_0.040IN  [TESTPOINT_0.040IN]
VSOL+  TEST_POINT_0.040IN  [TESTPOINT_0.040IN]
VSOL-  TEST_POINT_0.040IN  [TESTPOINT_0.040IN]

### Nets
3V3: 3V3.TESTPOINT ; also sheet 2,7
5V_1: 5V_1.TESTPOINT ; also sheet 3,7
5V_2: 5V_2.TESTPOINT ; also sheet 4,7
5V_3: 5V_3.TESTPOINT ; also sheet 5,8
5V_4: 5V_4.TESTPOINT ; also sheet 6,8
!INT: !INT.TESTPOINT ; also sheet 1,7,8
GND: GND.TESTPOINT ; also sheet 1,2,3,4,5,6,7,8
SCL: SCL.TESTPOINT ; also sheet 1,7,8
SDA: SDA.TESTPOINT ; also sheet 1,7,8
VBATT: VBATT.TESTPOINT ; also sheet 1,2,3,4,5,6
VCC_BACKPLANE: BACK.TESTPOINT ; also sheet 1,7,8
VCC_LINUX: LINUX.TESTPOINT ; also sheet 1,7
VCC_MOD0: MOD0.TESTPOINT ; also sheet 1,7
VCC_MOD1: MOD1.TESTPOINT ; also sheet 1,7
VCC_MOD2: MOD2.TESTPOINT ; also sheet 1,8
VCC_MOD5: MOD5.TESTPOINT ; also sheet 1,8
VCC_MOD6: MOD6.TESTPOINT ; also sheet 1,8
VCC_MOD7: MOD7.TESTPOINT ; also sheet 1,8
VSOL+: VSOL+.TESTPOINT ; also sheet 1
VSOL-: VSOL-.TESTPOINT ; also sheet 1

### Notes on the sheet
- Debugging

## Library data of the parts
3V3 5V_1-5V_4 !INT BACK GND LINUX MOD0 MOD1 MOD2 MOD5-MOD7 SCL SDA VBATT VSOL+ VSOL- = headers:TEST_POINT_0.040IN: 0.040in Test Point; DIGIKEY: 5001K-ND
C1-C28 = passives:CAPACITOR: 0402 Capacitor
J1 = signpost:MODULE_POWER: Header for power module for signpost; DIGIKEY: S9172-ND
JP1 JP2 = SparkFun-Connectors:M02: Header 2
L1-L5 = passives:INDUCTOR: A very specific inductor; DIGIKEY: 541-1322-1-ND
R1-R47 = passives:RESISTOR: Resistor
U1-U5 = chips:TLV62130: High Efficient 3A switching step-down regulator. 1V-5V out, 4V-17V in.; DIGIKEY: 296-35978-1-ND
U6 U7 = signpost:PCA9544A: 1-4 I2C/SMBUS Multiplexer with interrupt for power supply coulomb counters; DIGIKEY: 296-20960-1-ND
U8-U15 = signpost:LTC2941: I2C Battery Gas Gauge with External Sense Resistor; DIGIKEY: LTC2941IDCB#TRMPBFCT-ND

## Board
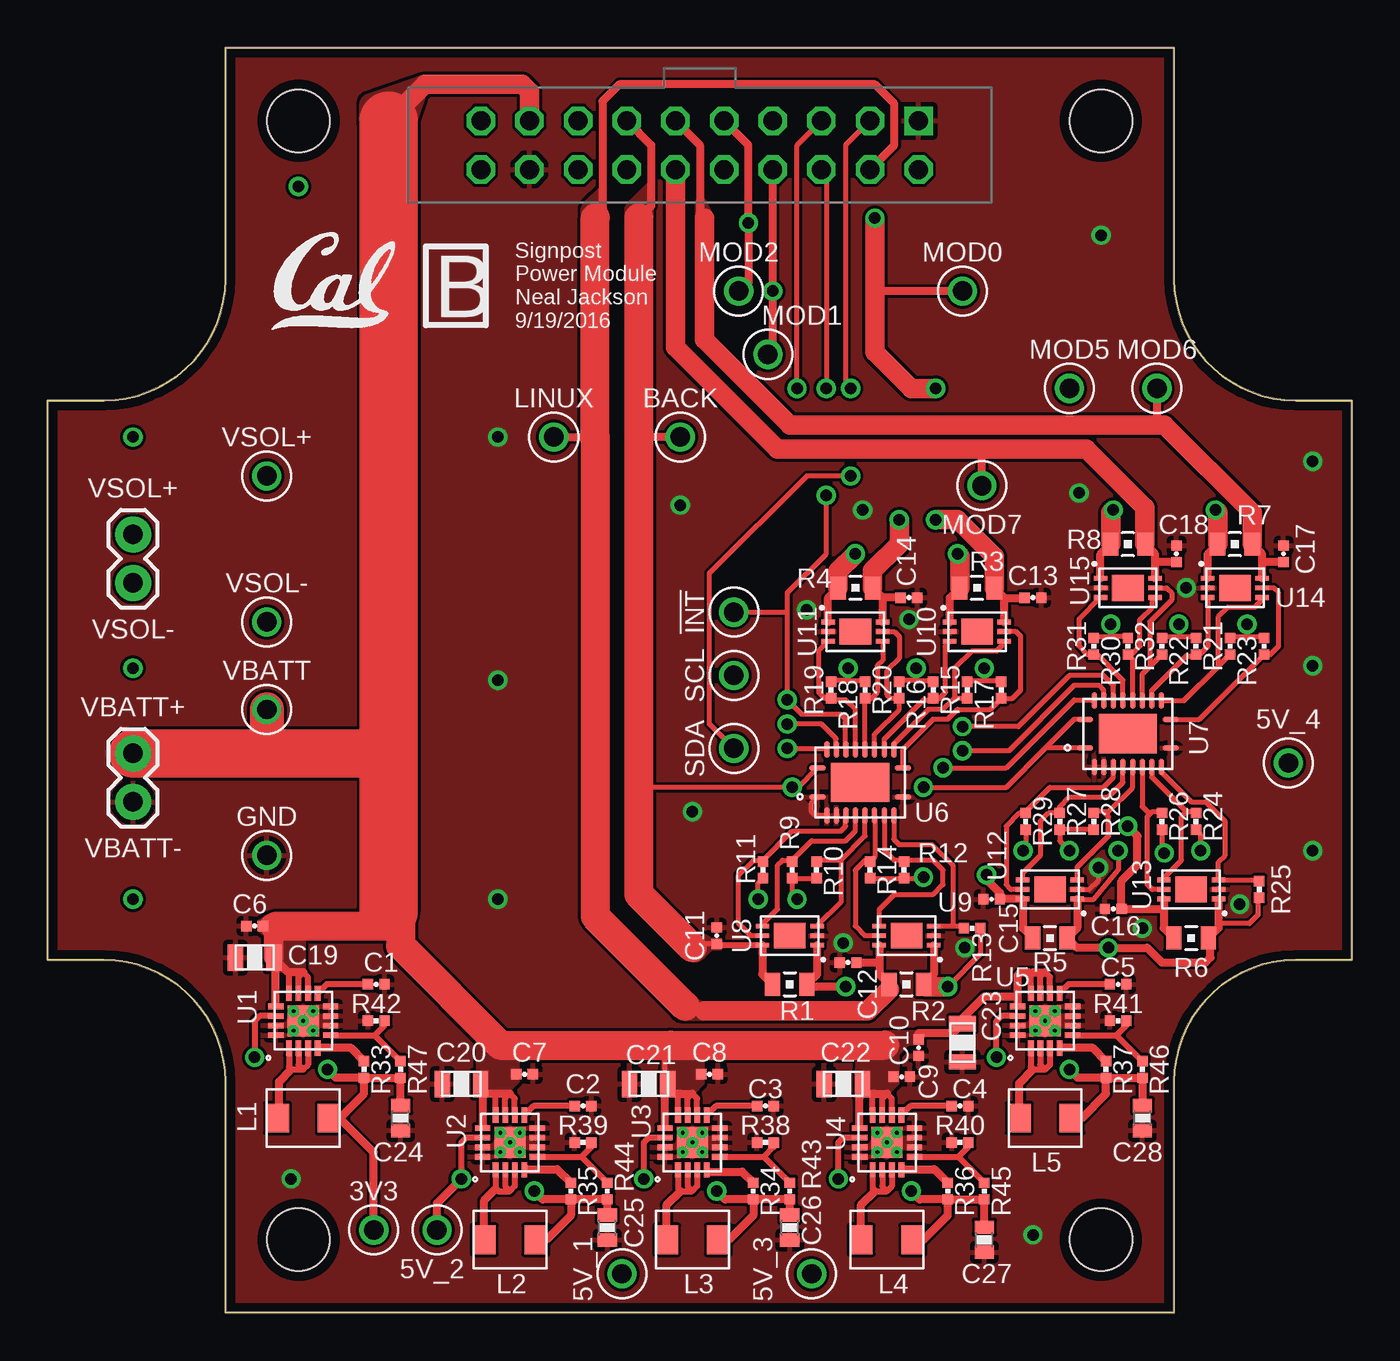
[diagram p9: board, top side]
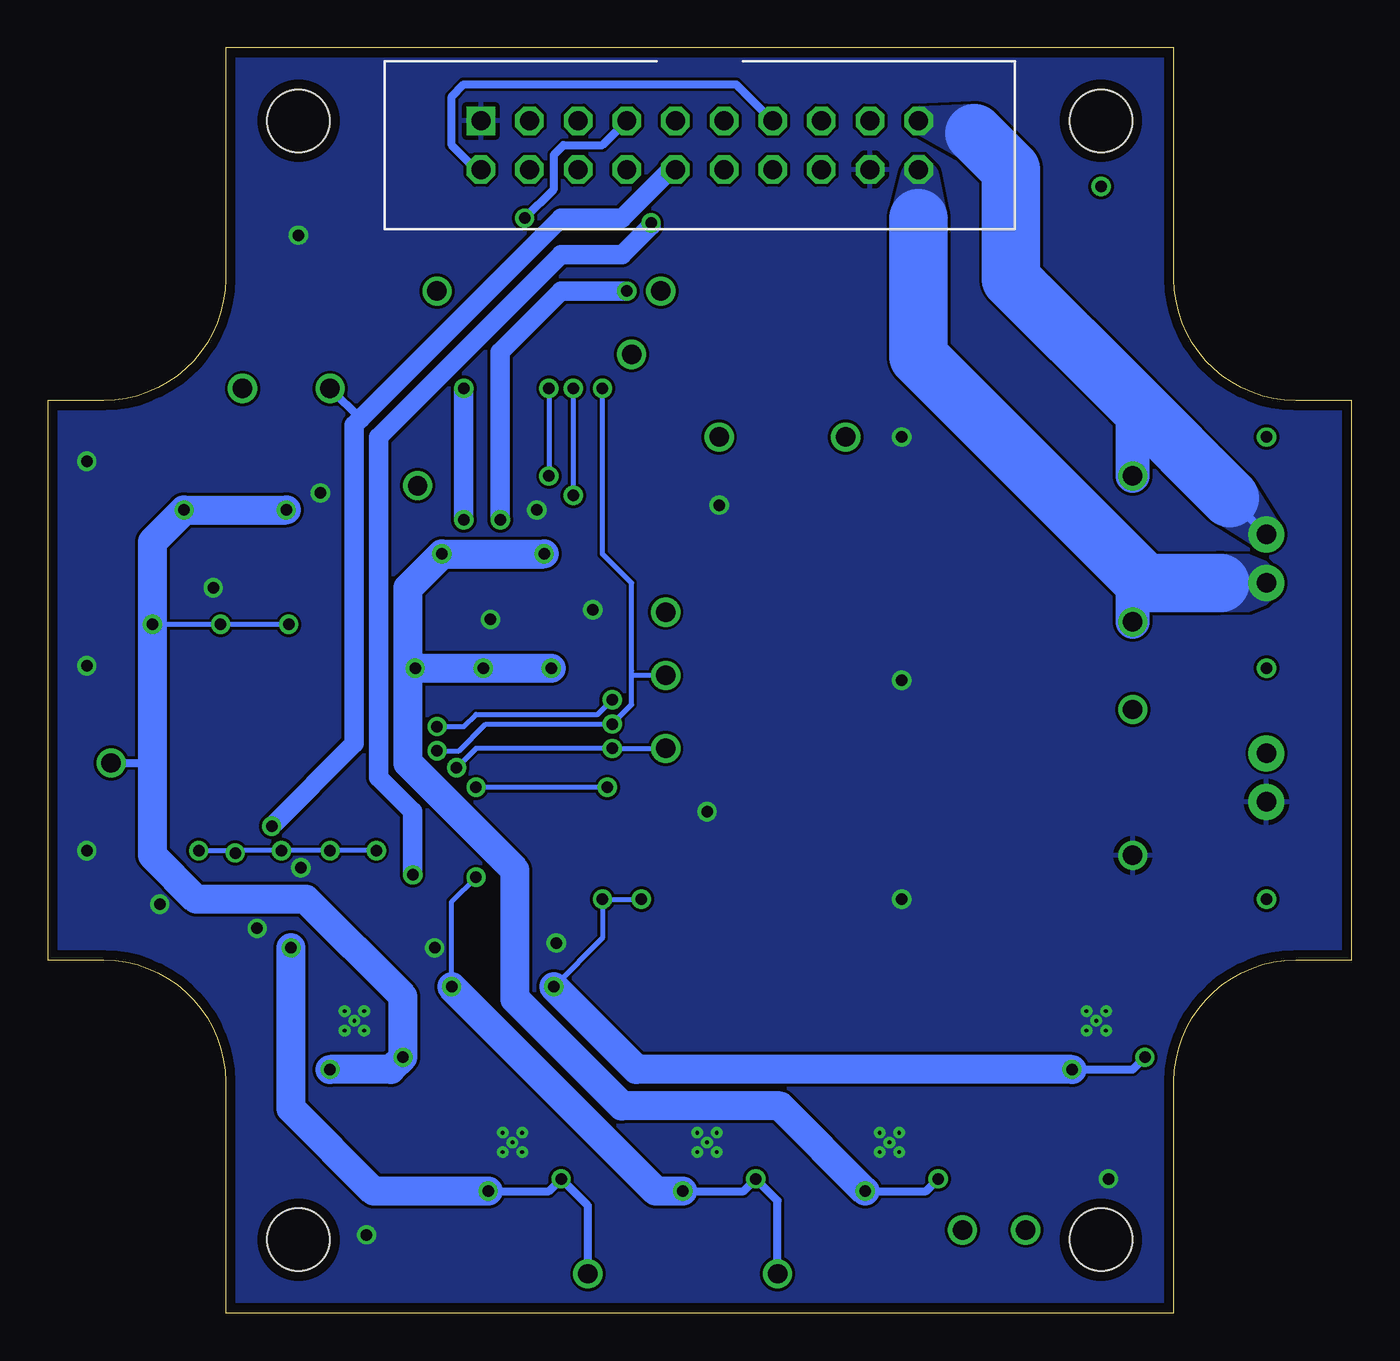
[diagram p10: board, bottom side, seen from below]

Size 68.07 x 66.04 mm. Coordinates in mm from the lower left corner, seen from the top.
Outline: 9.27,0 9.27,12.06 arc90 2.92,18.41 0,18.41 0,47.62 2.92,47.62 arc90 9.27,53.98 9.27,66.04 58.8,66.04 58.8,53.98 arc90 65.15,47.62 68.07,47.62 68.07,18.41 65.15,18.41 arc90 58.8,12.06 58.8,0 9.27,0
Copper layers (1*16): Top 0.0178mm / dielectric 59mil / Bottom 0.0178mm
Design rules "sunstone-2lyr_v1.0.0.3 *": minimum track width 6mil, minimum drill 14mil, track to track 6mil, track to pad 6mil, pad to pad 6mil, via to via 6mil, smd to smd 6mil, copper to edge 20mil, drill to drill 16mil, minimum pad ring 8mil, minimum via ring 8mil, stop-mask expansion 3mil, vias tented up to drill 30mil, thermal gap 10mil
Holes 3.26 mm at 13.08,62.23 54.99,62.23 13.08,3.81 54.99,3.81

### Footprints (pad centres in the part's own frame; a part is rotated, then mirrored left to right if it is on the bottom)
TESTPOINT_0.040IN = drill 1.016: TESTPOINT 0,0
0402_CAP = smd 0.536 x 0.546: 1 -0.433,0; 2 0.433,0
0805_CAP = smd 0.8 x 1.4: P$1 1,0; P$2 -1,0
0603_CAP = smd 0.7 x 1: 1 -0.65,0; 2 0.65,0
MODULE_POWER = drill 0.991 square: 1 11.43,29.21 | drill 0.991 octagon: 2 11.43,26.67; 3 8.89,29.21; 4 8.89,26.67; 5 6.35,29.21; 6 6.35,26.67; 7 3.81,29.21; 8 3.81,26.67; 9 1.27,29.21; 10 1.27,26.67; 11 -1.27,29.21; 12 -1.27,26.67; 13 -3.81,29.21; 14 -3.81,26.67; 15 -6.35,29.21; 16 -6.35,26.67; 17 -8.89,29.21; 18 -8.89,26.67; 19 -11.43,29.21; 20 -11.43,26.67
1X02 = drill 1.016 pad 1.88: 1 0,0; 2 2.54,0
IHL-1212BZ-11 = smd 1.2 x 1.5: P$1 -1.35,0; P$2 1.35,0
0805_RES = smd 0.8 x 1.2: 1 -0.9,0; 2 0.9,0
0402_RES = smd 0.536 x 0.546: 1 -0.433,0; 2 0.433,0
TQFN-16/3MM = smd 0.3 x 0.8: 1 -0.75,-1.43; 2 -0.25,-1.43; 3 0.25,-1.43; 4 0.75,-1.43; 9 0.75,1.43; 10 0.25,1.43; 11 -0.25,1.43; 12 -0.75,1.43 | smd 0.8 x 0.3: 5 1.43,-0.75; 6 1.43,-0.25; 7 1.43,0.25; 8 1.43,0.75; 13 -1.43,0.75; 14 -1.43,0.25; 15 -1.43,-0.25; 16 -1.43,-0.75 | smd 1.63 x 1.63: GND 0,0
QFN-N20 = smd 0.85 x 0.28: 1 -2.23,-0.75; 10 2.23,-0.75; 11 2.23,0.75; 20 -2.23,0.75 | smd 0.28 x 0.85: 2 -1.75,-1.73; 3 -1.25,-1.73; 4 -0.75,-1.73; 5 -0.25,-1.73; 6 0.25,-1.73; 7 0.75,-1.73; 8 1.25,-1.73; 9 1.75,-1.73; 12 1.75,1.73; 13 1.25,1.73; 14 0.75,1.73; 15 0.25,1.73; 16 -0.25,1.73; 17 -0.75,1.73; 18 -1.25,1.73; 19 -1.75,1.73 | smd 3.05 x 2.05: P$22 0,0
DFN-6-2MMX3MM = smd 0.25 x 0.7: 1 -0.5,-1.425; 2 0,-1.425; 3 0.5,-1.425; 4 0.5,1.425; 5 0,1.425; 6 -0.5,1.425 | smd 1.35 x 1.65: NC 0,0

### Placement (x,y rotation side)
3V3  17.02,4.32 0 top
5V_1  29.97,2.03 0 top
5V_2  20.32,4.32 0 top
5V_3  39.88,2.03 0 top
5V_4  64.77,28.7 0 top
!INT  35.81,36.58 0 top
BACK  33.02,45.72 0 top
C1  17.14,17.14 180 top
C2  27.94,10.79 180 top
C3  37.47,10.79 180 top
C4  47.62,10.79 180 top
C5  55.88,17.14 180 top
C6  10.79,20.19 180 top
C7  24.89,12.45 0 top
C8  34.54,12.45 0 top
C9  44.58,12.32 0 top
C10  45.47,13.84 270 top
C11  34.92,19.68 90 top
C12  41.78,18.29 180 top
C13  51.44,37.34 0 top
C14  44.96,37.34 0 top
C15  49.28,21.59 180 top
C16  55.63,21.08 180 top
C17  64.52,39.62 90 top
C18  58.93,39.62 90 top
C19  10.79,18.54 0 top
C20  21.59,11.94 0 top
C21  31.37,11.94 0 top
C22  41.53,11.94 0 top
C23  47.75,14.1 90 top
C24  18.41,10.16 90 top
C25  29.21,4.45 90 top
C26  38.73,4.45 90 top
C27  48.9,3.81 90 top
C28  57.15,10.16 90 top
GND  11.43,23.88 0 top
J1  34.04,33.02 0 top
JP1  4.45,38.1 90 top
JP2  4.45,26.67 90 top
L1  13.34,10.16 0 top
L2  24.13,3.81 0 top
L3  33.66,3.81 0 top
L4  43.81,3.81 0 top
L5  52.07,10.16 0 top
LINUX  26.42,45.72 0 top
MOD0  47.75,53.34 270 top
MOD1  37.59,50.04 0 top
MOD2  36.07,53.34 0 top
MOD5  53.34,48.26 0 top
MOD6  57.91,48.26 0 top
MOD7  48.77,43.18 0 top
R1  38.73,17.14 0 top
R2  44.83,17.14 0 top
R3  48.51,37.85 180 top
R4  42.16,37.85 180 top
R5  52.32,19.56 0 top
R6  59.69,19.56 0 top
R7  61.98,40.13 180 top
R8  56.39,40.13 180 top
R9  38.86,23.11 270 top
R10  40.13,23.11 270 top
R11  37.34,23.11 270 top
R12  44.7,23.11 270 top
R13  48.26,20.07 0 top
R14  42.93,23.11 270 top
R15  48.01,32.51 90 top
R16  46.23,32.51 90 top
R17  49.78,32.51 90 top
R18  42.67,32.51 90 top
R19  40.89,32.51 90 top
R20  44.45,32.51 90 top
R21  61.72,34.8 90 top
R22  59.94,34.8 90 top
R23  63.5,34.8 90 top
R24  59.94,25.65 270 top
R25  63.25,22.1 270 top
R26  58.17,25.65 270 top
R27  52.83,25.65 270 top
R28  54.61,25.65 270 top
R29  51.05,25.65 270 top
R30  56.39,34.8 90 top
R31  54.61,34.8 90 top
R32  58.17,34.8 90 top
R33  16.51,12.7 270 top
R34  36.83,6.35 270 top
R35  27.3,6.35 270 top
R36  46.99,6.35 270 top
R37  55.24,12.7 270 top
R38  37.47,8.89 0 top
R39  27.94,8.89 0 top
R40  47.62,8.89 0 top
R41  55.88,15.24 0 top
R42  17.14,15.24 0 top
R43  38.73,6.35 270 top
R44  29.21,6.35 270 top
R45  48.9,6.35 270 top
R46  57.15,12.7 270 top
R47  18.41,12.7 270 top
SCL  35.81,33.27 0 top
SDA  35.81,29.46 0 top
U1  13.34,15.24 0 top
U2  24.13,8.89 0 top
U3  33.66,8.89 0 top
U4  43.81,8.89 0 top
U5  52.07,15.24 0 top
U6  42.42,27.69 0 top
U7  56.39,30.23 0 top
U8  38.73,19.68 90 top
U9  44.83,19.68 90 top
U10  48.51,35.56 270 top
U11  42.16,35.56 270 top
U12  52.32,22.1 90 top
U13  59.69,22.1 90 top
U14  61.98,37.85 270 top
U15  56.39,37.85 270 top
U$1  [UCB_CAL_200MIL]  11.68,51.31 0 top
VBATT  11.43,31.5 0 top
VSOL+  11.43,43.69 0 top
VSOL-  11.43,36.07 0 top

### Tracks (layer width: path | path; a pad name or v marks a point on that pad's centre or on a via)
3V3  (via drill 0.6)
  Top 0.254: v37.08,21.59 37.08,22.43 R11.2 | v39.12,21.59 38.86,21.84 R9.2 R10.2
  Top 0.305: U1.14 11.04,15.49 10.79,15.24 v10.79,13.34
  Top 0.406: L1.P$2 15.24,10.16 | 15.24,10.16 16.51,11.43 R33.2 | R33.2 R47.2 C24.2 | R33.2 15.04,12.27 v14.61,12.7 | U8.1 40.16,17.67 R1.2 39.76,17.02 v41.66,17.02 | 3V3.TESTPOINT 17.02,8.38 15.24,10.16
  Bottom 0.254: v37.08,21.59 v39.12,21.59 39.12,19.56 v41.66,17.02
  Bottom 0.406: v14.61,12.7 11.43,12.7 v10.79,13.34
  Bottom 1.524: v14.61,12.7 37.34,12.7 v41.66,17.02
5V_1  (via drill 0.6)
  Top 0.254: R14.2 R12.2 45.67,22.68 v45.72,22.73 | R13.2 48.69,18.72 v46.99,17.02
  Top 0.305: v31.11,6.99 31.11,8.89 31.36,9.14 U3.14
  Top 0.406: R34.2 R43.2 C26.2 | R34.2 35.36,5.92 v34.92,6.35 | R34.2 36.83,5.08 35.56,3.81 L3.P$2 | U9.1 46.26,17.67 R2.2 45.86,17.02
  Top 1.016: v46.99,17.02 45.86,17.02
  Bottom 0.254: v46.99,17.02 46.99,21.46 v45.72,22.73
  Bottom 0.406: v34.92,6.35 31.75,6.35 v31.11,6.99 29.97,5.84 5V_1.TESTPOINT
  Bottom 1.524: v34.92,6.35 36.32,6.35 v46.99,17.02
5V_2  (via drill 0.6)
  Top 0.254: v48.9,33.66 48.9,33.02 | 48.9,33.02 49.71,33.02 R17.2 | R15.2 48.01,33.02 48.9,33.02 | v45.34,33.66 45.34,33.02 | 45.34,33.02 46.15,33.02 R16.2 | 45.34,33.02 44.52,33.02 R20.2 | U10.1 | v41.78,33.66 41.78,33.02 | 41.78,33.02 42.6,33.02 R18.2 | 41.78,33.02 40.97,33.02 R19.2
  Top 0.305: v21.59,6.99 21.59,8.89 21.84,9.14 U2.14
  Top 0.406: R35.2 27.3,5.08 26.04,3.81 L2.P$2 | R35.2 R44.2 C25.2 | R35.2 25.83,5.92 v25.4,6.35 | v21.59,6.99 20.32,5.71 5V_2.TESTPOINT | U10.1 47.09,37.32 R3.2 | U11.1 40.74,37.32 R4.2
  Top 1.016: R3.2 47.61,39.51 v47.5,39.62 | R4.2 41.26,38.72 v42.16,39.62
  Bottom 0.406: v25.4,6.35 22.23,6.35 v21.59,6.99 | v48.9,33.66 48.77,33.53
  Bottom 1.524: v25.4,6.35 29.84,10.79 38.1,10.79 43.69,16.38 43.69,23.11 49.28,28.7 49.28,33.78 | v41.78,33.66 v45.34,33.66 v48.9,33.66 49.15,33.66 49.28,33.78 | 49.28,33.78 49.28,37.85 v47.5,39.62 v42.16,39.62
5V_3  (via drill 0.6)
  Top 0.254: U12.1 54.61,21.59 55.88,23.11 v55.88,24.13 | R29.2 51.05,24.26 v50.93,24.13 | R28.2 R27.2 52.83,24.64 v53.34,24.13 | R26.2 58.17,24.13 v58.29,24 | v60.2,24.13 60.2,24.97 R24.2 | R25.2 63.18,21.6 63.18,20.76 62.74,20.32 61.12,20.32
  Top 0.305: v41.27,6.99 41.27,8.89 41.52,9.14 U4.14
  Top 0.406: C27.2 R45.2 R36.2 | L4.P$2 45.72,3.81 46.99,5.08 R36.2 | R36.2 45.52,5.92 v45.09,6.35 | U12.1 53.75,20.08 R5.2 53.73,19.05 v55.37,19.05 57.4,19.05 58.17,18.29 60.45,18.29 60.71,18.54 60.71,19.44 R6.2 | 60.71,19.67 R6.2 | U13.1 61.12,20.32 61.12,20.08 R6.2
  Bottom 0.254: v60.2,24.13 58.42,24.13 v58.29,24 58.17,24.13 v55.88,24.13 v53.34,24.13 v50.93,24.13
  Bottom 0.406: v45.09,6.35 41.91,6.35 v41.27,6.99 39.88,5.59 5V_3.TESTPOINT
  Bottom 1.524: v45.09,6.35 51.05,6.35 55.37,10.67 v55.37,19.05
5V_4  (via drill 0.6)
  Top 0.254: R30.2 56.39,35.31 55.5,35.31 | 55.5,35.31 v55.5,35.94 | R31.2 54.66,35.23 54.74,35.31 55.5,35.31 | R32.2 58.22,35.23 58.29,35.31 59.05,35.31 | v59.05,35.94 59.05,35.31 | 59.05,35.31 59.87,35.31 R22.2 | R21.2 61.77,35.23 61.85,35.31 62.61,35.31 | 62.61,35.31 63.42,35.31 R23.2 | v62.61,35.94 62.61,35.31 | U14.1
  Top 0.305: v49.53,13.34 49.53,15.24 49.78,15.49 U5.14
  Top 0.406: R37.2 R46.2 C28.2 | R37.2 53.77,12.27 v53.34,12.7 | L5.P$2 53.98,10.16 55.24,11.43 R37.2 | U15.1 54.96,39.61 R8.2 | U14.1 60.55,39.61 R7.2
  Top 1.016: R8.2 55.49,41.77 v55.63,41.91 | R7.2 61.08,41.79 v60.96,41.91
  Bottom 0.254: v55.5,35.94 v59.05,35.94 v62.61,35.94
  Bottom 0.406: 5V_4.TESTPOINT 62.61,28.7
  Bottom 1.524: v53.34,12.7 50.16,12.7 v49.53,13.34 49.53,16.51 54.61,21.59 60.33,21.59 62.61,23.88 62.61,28.7 v62.61,35.94 62.61,40.26 v60.96,41.91 v55.63,41.91
!INT  (via drill 0.6)
  Top 0.254: J1.6 40.64,59.44 v40.64,48.26 | U7.17 55.64,32.75 55.12,33.27 53.34,33.27 50.67,30.61 v47.75,30.61 | U6.17 41.66,29.43 41.66,30.99 41.4,31.24 39.37,31.24 v38.61,32 38.61,36.58 | 38.61,36.58 38.61,37.59 40.64,39.62 v40.64,42.67 | !INT.TESTPOINT 38.61,36.58
  Bottom 0.254: v40.64,48.26 v40.64,42.67 | v47.75,30.61 46.35,30.61 45.72,31.24 39.37,31.24 v38.61,32
GND  (via drill 0.2, 0.6)
  Top 0.254: U12.2 54.36,22.1 54.86,22.61 v54.86,23.24 | U6.2 40.08,25.96 39.88,26.16 39.88,26.63 U6.1
  other vias: 54.99,56.26 12.83,15.75 13.84,15.75 13.34,15.24 12.83,14.73 13.84,14.73 24.13,8.89 23.62,9.4 24.64,9.4 23.62,8.38 24.64,8.38 33.66,8.89 33.15,9.4 34.16,9.4 34.16,8.38 33.15,8.38 43.81,8.89 43.31,8.38 44.32,8.38 44.32,9.4 43.31,9.4 52.07,15.24 51.56,15.75 52.58,15.75 52.58,14.73 51.56,14.73 66.04,44.45 53.85,42.8 42.55,41.91 23.5,45.72 33.02,42.16 33.66,26.16 66.04,33.78 23.5,21.59 12.7,6.99 51.44,4.06 66.04,24.13 23.5,33.02 41.53,19.3 57.15,20.07 44.96,36.2 47.88,19.05 62.23,21.34 39.62,36.7 59.44,37.85
  pour Top (rank 2): -1.27,67.31 68.58,67.31 68.58,-1.27 -1.27,-1.27
  pour Bottom (rank 2): -1.27,67.31 68.58,67.31 68.58,-1.27 -1.27,-1.27
N$1
  Top 0.305: C2.2 25.36,10.79 U2.9
N$2
  Top 0.305: U2.1 23.38,6.46 23.5,6.35 24.13,6.35 | U2.3 24.38,6.6 24.13,6.35 | U2.2 23.88,6.6 24.13,6.35
  Top 0.406: L2.P$1 22.78,5.87 23.38,6.46
N$3
  Top 0.305: U2.4 24.99,7.46 25.02,7.49
  Top 0.406: 25.02,7.49 26.59,7.49 R35.1
N$4
  Top 0.305: U2.5 27.85,8.14 | 27.85,8.14 R44.1 | R39.2 28.37,8.66 27.85,8.14
N$5
  Top 0.305: C3.2 34.88,10.79 U3.9
N$6
  Top 0.305: U3.1 32.91,6.46 33.02,6.35 33.66,6.35 | U3.2 33.41,6.6 33.66,6.35 | U3.3 33.91,6.6 33.66,6.35
  Top 0.406: L3.P$1 32.3,5.63 33.02,6.35
N$7
  Top 0.305: U3.4 34.45,7.46 34.54,7.37
  Top 0.406: 34.54,7.37 36.25,7.37 R34.1
N$8
  Top 0.305: C4.2 45.04,10.79 U4.9
N$9
  Top 0.305: U3.5 37.38,8.14 | 37.38,8.14 R43.1 | R38.2 37.9,8.66 37.38,8.14
N$10
  Top 0.305: U4.1 43.06,6.46 43.18,6.35 43.81,6.35 | U4.3 44.06,6.6 43.81,6.35 | U4.2 43.56,6.6 43.81,6.35
  Top 0.406: L4.P$1 42.47,5.63 43.18,6.35
N$11
  Top 0.305: U4.4 44.67,7.46 44.7,7.49
  Top 0.406: 44.7,7.49 46.28,7.49 R36.1
N$12
  Top 0.305: U4.5 47.54,8.14 | 47.54,8.14 R45.1 | R40.2 48.06,8.66 47.54,8.14
N$13
  Top 0.305: C5.2 53.3,17.14 U5.9
N$14
  Top 0.305: U5.1 51.32,12.81 51.44,12.7 52.07,12.7 | U5.3 52.32,12.95 52.07,12.7 | U5.2 51.82,12.95 52.07,12.7
  Top 0.406: L5.P$1 50.72,11.98 51.44,12.7
N$15
  Top 0.305: U5.4 52.93,13.81 52.96,13.84
  Top 0.406: 52.96,13.84 54.53,13.84 R37.1
N$16
  Top 0.305: U5.5 55.79,14.49 | 55.79,14.49 R46.1 | R41.2 56.31,15.01 55.79,14.49
N$20  (via drill 0.6)
  other vias: 4.45,45.72
N$21
  Top 0.254: U12.4 50.9,22.96 51.82,23.88 51.82,25.65 52.25,26.09 R27.1 52.83,26.42 53.34,26.92 55.37,26.92 56.13,27.69 U7.5
N$22
  Top 0.254: U12.3 53.75,23.27 55.37,24.89 55.37,25.91 55.12,26.16 | 55.12,26.16 54.69,26.16 R28.1 | 55.12,26.16 55.37,26.16 56.64,27.43 U7.6
N$23
  Top 0.254: U7.12 59.31,31.96 61.05,33.69 61.09,33.73 | 61.09,33.73 R21.1 | U14.4 63.4,37.24 62.99,36.83 61.59,36.83 61.09,36.32 61.09,33.73
N$24
  Top 0.254: U7.13 57.64,32.49 59.44,34.29 59.87,34.29 R22.1 60.15,34.37 60.58,34.8 60.58,37.32 U14.3
N$25
  Top 0.254: U7.11 60.11,30.98 R23.1 63.83,34.37 64.26,34.8 64.26,37.59 64.01,37.85 U14.5
N$26
  Top 0.254: U7.15 56.64,34.11 R30.1 56.59,34.37 57.02,34.8 57.02,36.2 57.66,36.83 57.66,37.19 U15.4
N$27
  Top 0.254: U7.16 56.14,33.02 54.79,34.37 R31.1 54.28,34.37 53.85,34.8 53.85,36.23 U15.3
N$28  (via drill 0.6)
  other vias: 4.45,33.66
N$29  (via drill 0.6)
  other vias: 4.45,21.59
N$30  (via drill 0.6)
  other vias: 13.08,58.8
N$43
  Top 0.254: U8.4 37.31,20.29 38.1,21.08 38.1,23.37 38.35,23.62 38.79,23.62 R9.1 38.86,23.62 39.88,24.64 41.66,24.64 42.16,25.15 U6.5
N$46
  Top 0.254: U7.14 57.14,33.34 57.37,33.56 57.53,33.73 | 57.53,33.73 R32.1 | U15.5 58.42,37.85 58.67,37.59 58.67,37.21 57.53,36.07 57.53,33.73
N$47
  Top 0.254: 41.4,23.62 40.21,23.62 R10.1 | U8.3 41.4,21.42 41.4,23.62 | 41.4,23.62 42.67,24.89 U6.6
N$48
  Top 0.254: U12.5 50.29,22.1 50.04,22.35 50.04,25.4 50.73,26.09 R29.1 51.05,26.16 52.32,27.43 55.12,27.43 55.63,27.94 55.63,28.48 U7.4
N$49
  Top 0.254: U13.4 58.27,22.7 59.18,23.62 59.18,25.91 59.44,26.16 | 59.44,26.16 59.87,26.16 R24.1 | U7.8 57.64,27.96 59.44,26.16
N$50
  Top 0.254: U7.9 58.14,28.22 59.69,26.67 60.45,26.67 61.47,25.65 61.47,23.88 61.12,23.52 U13.3 63.18,22.6 R25.1
N$51
  Top 0.254: U13.5 57.66,22.1 57.4,22.35 57.4,25.91 57.53,26.04 | 57.53,26.04 57.66,26.16 58.09,26.16 R26.1 | U7.7 57.14,26.43 57.53,26.04
N$52
  Top 0.254: U10.4 49.94,34.95 49.53,34.54 48.26,34.54 47.37,33.66 47.37,32 | R15.1 47.45,32.08 47.37,32 | 47.37,32 47.24,32 46.74,31.5 45.97,31.5 44.17,29.69 U6.12
N$53
  Top 0.254: U10.3 46.86,34.83 46.86,32.38 46.56,32.08 R16.1 46.15,32 45.72,32 43.67,29.95 U6.13
N$54
  Top 0.254: R17.1 49.71,32 49.71,31.93 | R17.1 50.37,32.08 50.8,32.51 50.8,35.31 50.55,35.56 U10.5 | U6.11 44.65,29.41 46.23,30.99 46.99,30.99 47.5,31.5 49.2,31.5 R17.1
N$55
  Top 0.254: U11.4 43.59,34.06 43.31,33.78 43.31,32.38 43,32.08 R18.1 U6.15
N$56
  Top 0.254: U11.3 40.26,34.58 40.26,32.38 40.56,32.08 R19.1 40.97,32 41.66,32 42.16,31.5 U6.16
N$57
  Top 0.254: U11.5 44.2,35.56 44.45,35.31 44.45,34.16 43.81,33.53 43.81,32.26 43.99,32.08 R20.1 44.45,31.5 43.17,30.21 U6.14
N$61
  Top 0.305: C1.2 14.56,17.14 U1.9
N$62
  Top 0.305: 12.06,10.24 L1.P$1 | U1.3 13.59,12.95 13.34,12.7 | U1.2 13.09,12.95 13.34,12.7 | U1.1 12.59,12.81 12.7,12.7 13.34,12.7
  Top 0.406: 12.06,10.24 12.06,12.06 12.7,12.7
N$63
  Top 0.305: U1.4 14.19,13.81 14.22,13.84
  Top 0.406: 14.22,13.84 15.8,13.84 R33.1
N$64
  Top 0.305: U1.5 17.06,14.49 | 17.06,14.49 R47.1 | R42.2 17.58,15.01 17.06,14.49
N$67
  Top 0.254: U8.5 36.7,19.68 36.07,20.32 36.07,22.86 36.83,23.62 37.26,23.62 R11.1 37.34,23.62 38.86,25.15 41.4,25.15 41.66,25.4 41.66,25.94 U6.4
N$68
  Top 0.254: U9.4 43.41,21.05 44.2,21.84 46.23,21.84 46.74,22.35 46.74,23.11 46.23,23.62 44.7,23.62 | 44.7,23.62 44.2,23.62 43.69,24.13 43.69,25.94 U6.8 | R12.1 44.7,23.62
N$70
  Top 0.254: 47.69,20.18 R13.1 47.71,20.18 47.24,20.18 | U9.3 47.24,20.18 | 47.24,20.18 47.24,23.37 46.18,24.43 44.45,24.43 | 44.45,24.43 44.42,24.43 | U6.9 44.17,24.71 44.45,24.43
N$71
  Top 0.254: U9.5 42.67,19.68 42.16,20.19 42.16,23.11 42.67,23.62 42.85,23.62 R14.1 43.18,23.8 43.18,25.94 U6.7
SCL  (via drill 0.6)
  Top 0.254: J1.5 39.12,60.96 v39.12,48.26 | U7.18 55.12,31.98 55.12,32.51 54.86,32.77 53.59,32.77 50.16,29.34 v47.75,29.34 | U6.18 41.15,29.44 41.15,29.97 40.39,30.73 v38.61,30.73
  Bottom 0.254: SCL.TESTPOINT 37.59,33.27 | 37.59,33.27 37.59,31.75 v38.61,30.73 45.21,30.73 46.61,29.34 v47.75,29.34 | v39.12,48.26 39.12,39.62 37.59,38.1 37.59,33.53 37.59,33.27
SDA  (via drill 0.6)
  Top 0.254: U7.19 54.59,32 53.59,32 50.04,28.45 v46.74,28.45 | J1.3 41.66,60.96 41.66,48.26 v41.91,48.26 | v38.61,29.46 40.62,29.46 U6.19 | v41.91,43.69 39.62,43.69 34.54,38.61 34.54,30.73 SDA.TESTPOINT
  Bottom 0.254: v46.74,28.45 45.72,29.46 v38.61,29.46 SDA.TESTPOINT | v41.91,48.26 v41.91,43.69
VBATT
  Top 0.254: U2.13 22.7,9.75 22.73,9.78 | 23.38,11.31 23.38,11.4 23.35,11.43 | 32.23,11.79 32.23,13.68 32.51,13.97
  Top 0.305: U1.13 11.9,16.04 | 12.59,17.26 U1.12 12.59,17.66 12.7,17.78 | U1.11 13.09,17.53 13.34,17.78 13.59,17.53 U1.10 | U2.10 24.38,11.18 24.13,11.43 23.88,11.18 U2.11 | U2.12 23.38,11.31 23.5,11.43 | U3.10 33.91,11.18 33.66,11.43 33.41,11.18 U3.11 | U3.12 32.91,11.31 33.02,11.43 | U3.13 32.23,9.69 | U4.10 44.06,11.18 43.81,11.43 43.56,11.18 U4.11 | U4.12 43.06,11.31 43.18,11.43 | U4.13 42.38,9.69 | U5.10 52.32,17.53 52.07,17.78 51.82,17.53 U5.11 | U5.12 51.32,17.66 51.44,17.78 | U5.13 50.64,16.04
  Top 0.406: 33.66,11.43 33.02,11.43 32.23,11.43 | 43.81,11.43 43.18,11.43 42.43,11.43 | 51.44,17.78 52.07,17.78 | 50.64,16.04 50.64,16.51 | 50.64,16.51 50.64,17.62 50.8,17.78 51.2,17.78 51.32,17.66 | 50.64,16.51 48.9,16.51 47.75,15.37 C23.P$1 47.26,14.61 45.47,14.61 C10.1 | C6.1 11.7,20.19 | 42.38,9.69 42.38,11.22 42.43,11.43 | 42.43,11.43 C22.P$1 | 11.9,16.04 11.9,18.43 C19.P$1 12.56,17.78 12.7,17.78 13.34,17.78 | 11.79,20.05 11.94,20.19 | 24.13,11.43 23.35,11.43 22.73,11.43 | 22.73,12.05 C20.P$1 22.73,11.79 22.73,11.43 | 22.73,9.78 22.73,11.43 | 32.23,9.69 32.23,11.43 | 32.23,11.43 32.23,11.79 C21.P$1 | 18.41,20.95 17.78,20.95
  Top 1.016: J1.17 25.15,63.75 24.77,64.14 19.68,64.14 17.78,62.23 | C19.P$1 11.79,20.05
  Top 1.27: 18.41,20.95 18.41,20.32 18.29,20.19 | 11.7,20.19 11.94,20.19
  Top 1.524: 11.94,20.19 18.29,20.19 | 18.41,20.32 18.41,19.18 23.62,13.97 32.51,13.97 43.69,13.97
  Top 1.778: VBATT.TESTPOINT 11.43,29.21
  Top 2.54: JP2.2 11.43,29.21 17.78,29.21
  Top 3.048: 17.78,62.23 17.78,29.21 17.78,20.95
  pour Top (isolate 0.127): 16.26,62.23 16.26,63.05 arc-71 16.68,63.65 19.56,64.64 19.68,63.37 19.3,62.23 16.51,62.23
  pour Top (no thermals): 12.06,20.83 11.64,20.83 arc37 11.26,20.7 10.92,20.45 10.92,19.94 11.26,19.68 arc37 11.64,19.56 12.06,19.56
  pour Top (no thermals): 22.35,14.48 22.35,11.43 24,11.43 24.64,12.06 24.64,14.48
  pour Top (no thermals): 32,13.72 32,11.43 33.78,11.43 34.29,11.94 34.29,13.72
  pour Top (no thermals): 42.16,13.97 42.16,11.43 43.94,11.43 44.45,11.94 44.45,13.46 44.96,13.97 45.72,13.97 45.72,14.73 43.69,14.73
  pour Top (no thermals): 11.94,17.78 13.46,17.78 13.46,19.81 11.94,19.81
VCC_BACKPLANE  (via drill 0.6)
  Top 0.254: 30.86,28.19 30.87,28.21 30.87,28.44 30.86,28.45 | 30.87,30.98 30.86,30.99 | 30.87,28.94 30.86,28.96 | v45.72,27.43 50.04,27.43 52.08,29.48 | U7.20 54.15,30.99 53.59,30.99 52.08,29.48 | U7.1 52.08,29.48 | C11.1 33.86,19.25 33.66,19.05 | 30.86,27.43 v38.86,27.43 39.18,27.43 U6.20
  Top 0.305: U8.6 34.99,19.18
  Top 0.406: U8.6 37.31,17.67 R1.1 | J1.13 31.5,60.96 31.5,57.78 30.86,57.15 | C11.1 34.99,19.18 | BACK.TESTPOINT 31.11,45.72 30.86,45.97
  Top 1.524: 33.66,19.05 30.86,21.84 30.86,27.43 30.86,28.19 30.86,28.45 30.86,28.96 30.86,30.99 30.86,45.97 30.86,57.15
  Bottom 0.254: v38.86,27.43 v45.72,27.43
  Bottom 0.406: J1.2 45.72,59.69 46.99,60.96 46.99,63.5 46.35,64.14 32.13,64.14 J1.13
  pour Top (no thermals): 33.66,19.81 34.1,19.81 arc-34 34.45,19.71 34.67,19.56 35.18,19.56 35.18,18.92 34.67,18.92 34.22,18.47 arc-45 33.77,18.29 33.66,18.29
  pour Top: 30.1,57.15 30.1,57.52 arc-45 30.28,57.97 31.37,59.05 31.62,59.05 31.62,57.15
VCC_LINUX
  Top 0.406: 43.93,16.88 R2.1 43.41,17.67 43.41,18.29 | U9.6 43.41,18.29 | J1.4 44.2,60.96 44.2,63.12 43.18,64.14 29.84,64.14 28.96,63.25 28.96,57.53 28.57,57.15 | LINUX.TESTPOINT 28.57,45.72 | C12.1 43.41,18.29
  Top 1.016: 43.93,16.88 42.8,15.75 34.29,15.75
  Top 1.524: 28.57,57.15 28.57,45.72 28.57,20.7 33.27,16
  pour Top: 27.81,57.15 27.81,57.52 arc-45 28,57.97 28.83,58.8 29.3,57.37 arc-18 29.34,57.17 29.34,57.15
  pour Top: 34.29,16.26 arc-45 33.94,16.4 33.71,16.64 33.66,16.64 32.61,15.6 32.78,15.43 arc45 33.23,15.24 34.29,15.24
VCC_MOD0  (via drill 0.6)
  Top 0.406: U10.6 49.94,37.32 | 49.94,37.32 R3.1 | 49.94,37.32 50.98,37.32 C13.1 | MOD0.TESTPOINT 43.43,53.34 43.18,53.59
  Top 1.016: v46.35,48.26 45.09,48.26 43.18,50.16 43.18,53.59 v43.18,57.15 | v46.35,41.4 47.5,41.4 49.41,39.49 R3.1
  Bottom 0.406: J1.7 39.12,60.96 41.15,60.96 41.66,60.45 41.66,58.67 v43.18,57.15
  Bottom 1.016: v46.35,41.4 v46.35,48.26
VCC_MOD1  (via drill 0.6)
  Top 0.406: J1.8 v37.85,53.34 37.85,50.29 MOD1.TESTPOINT | U11.6 43.59,37.32 | 43.59,37.32 R4.1 | C14.1 43.61,37.34 43.59,37.32
  Top 1.016: R4.1 43.06,38.75 44.45,40.13 v44.45,41.4
  Bottom 1.016: v37.85,53.34 41.27,53.34 44.45,50.16 v44.45,41.4
VCC_MOD2  (via drill 0.6)
  Top 0.406: R5.1 50.9,20.08 U12.6 C15.1 49.71,21.92 49.02,22.61 v49.02,22.86 | J1.9 36.58,60.96 v36.58,56.9 36.58,53.72 MOD2.TESTPOINT
  Bottom 0.406: v36.58,56.9 36.58,56.77
  Bottom 1.016: 36.58,56.77 38.1,55.24 41.27,55.24 50.8,45.72 50.8,27.94 49.02,26.16 v49.02,22.86
VCC_MOD5  (via drill 0.6)
  Top 0.406: U13.6 58.27,21.08 | 58.27,21.08 58.27,20.08 R6.1 | 58.27,21.08 C16.1 56.06,22.53 56.9,23.37 56.9,24.89 v56.39,25.4
  Bottom 0.406: J1.10 35.56,59.69 | MOD5.TESTPOINT 51.75,46.67
  Bottom 1.016: 35.56,59.69 38.1,57.15 41.27,57.15 51.75,46.67 52.07,46.35 52.07,29.72 v56.39,25.4
VCC_MOD6
  Top 0.406: J1.11 34.04,60.96 34.04,57.4 34.29,57.15 | U14.6 63.4,39.12 | 63.4,39.12 63.4,39.61 R7.1 | C17.1 63.48,39.19 63.4,39.12 | MOD6.TESTPOINT 57.91,46.61 57.66,46.35
  Top 1.016: 34.29,57.15 34.29,50.8 38.73,46.35 57.66,46.35 58.29,46.35 62.88,41.77 R7.1
  pour Top: 33.78,57.15 33.78,57.72 arc-11 33.79,57.85 33.91,58.42 34.16,58.42 34.74,57.39 arc-29 34.8,57.15
VCC_MOD7
  Top 0.406: U15.6 57.81,39.12 | 57.81,39.12 57.81,39.61 R8.1 | C18.1 57.89,39.19 57.81,39.12 | MOD7.TESTPOINT 48.77,45.09
  Top 1.016: J1.12 32.77,50.42 38.1,45.09 48.77,45.09 54.23,45.09 57.29,42.03 R8.1
VSOL+
  Bottom 0.406: JP1.2 6.35,42.55
  Bottom 1.778: VSOL+.TESTPOINT 11.43,47.62
  Bottom 3.048: 19.68,61.59 17.78,59.69 17.78,53.98 11.43,47.62 6.35,42.55
  pour Bottom (no thermals): 7.11,41.27 5.08,43.31 3.81,41.27 3.81,40.01 5.08,40.01
  pour Bottom (no thermals): 22.61,62.99 19.68,63.12 19.68,60.33 20.57,60.33 22.61,61.47
VSOL-
  Bottom 1.778: VSOL-.TESTPOINT 11.43,37.47 10.79,38.1
  Bottom 3.048: 22.61,57.15 22.61,49.91 10.79,38.1 6.86,38.1
  pour Bottom (no thermals): 21.08,57.15 21.55,59.5 arc-34 21.73,59.83 22.35,60.45 22.86,60.45 23.4,59.8 arc-26 23.53,59.55 24.13,57.15
  pour Bottom (no thermals): 6.86,39.62 5.35,39.62 4.45,39.25 4.06,38.86 4.06,37.59 4.06,37.34 4.45,36.95 5.35,36.58 6.86,36.58

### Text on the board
tPlace: Signpost / Power Module / Neal Jackson / 9/19/2016 | B
tNames: VSOL+ | VSOL- | VBATT+ | VBATT-

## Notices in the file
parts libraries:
SparkFun-Connectors: Licensing: CC v3.0 Share-Alike You are welcome to use this library for commercial purposes.
